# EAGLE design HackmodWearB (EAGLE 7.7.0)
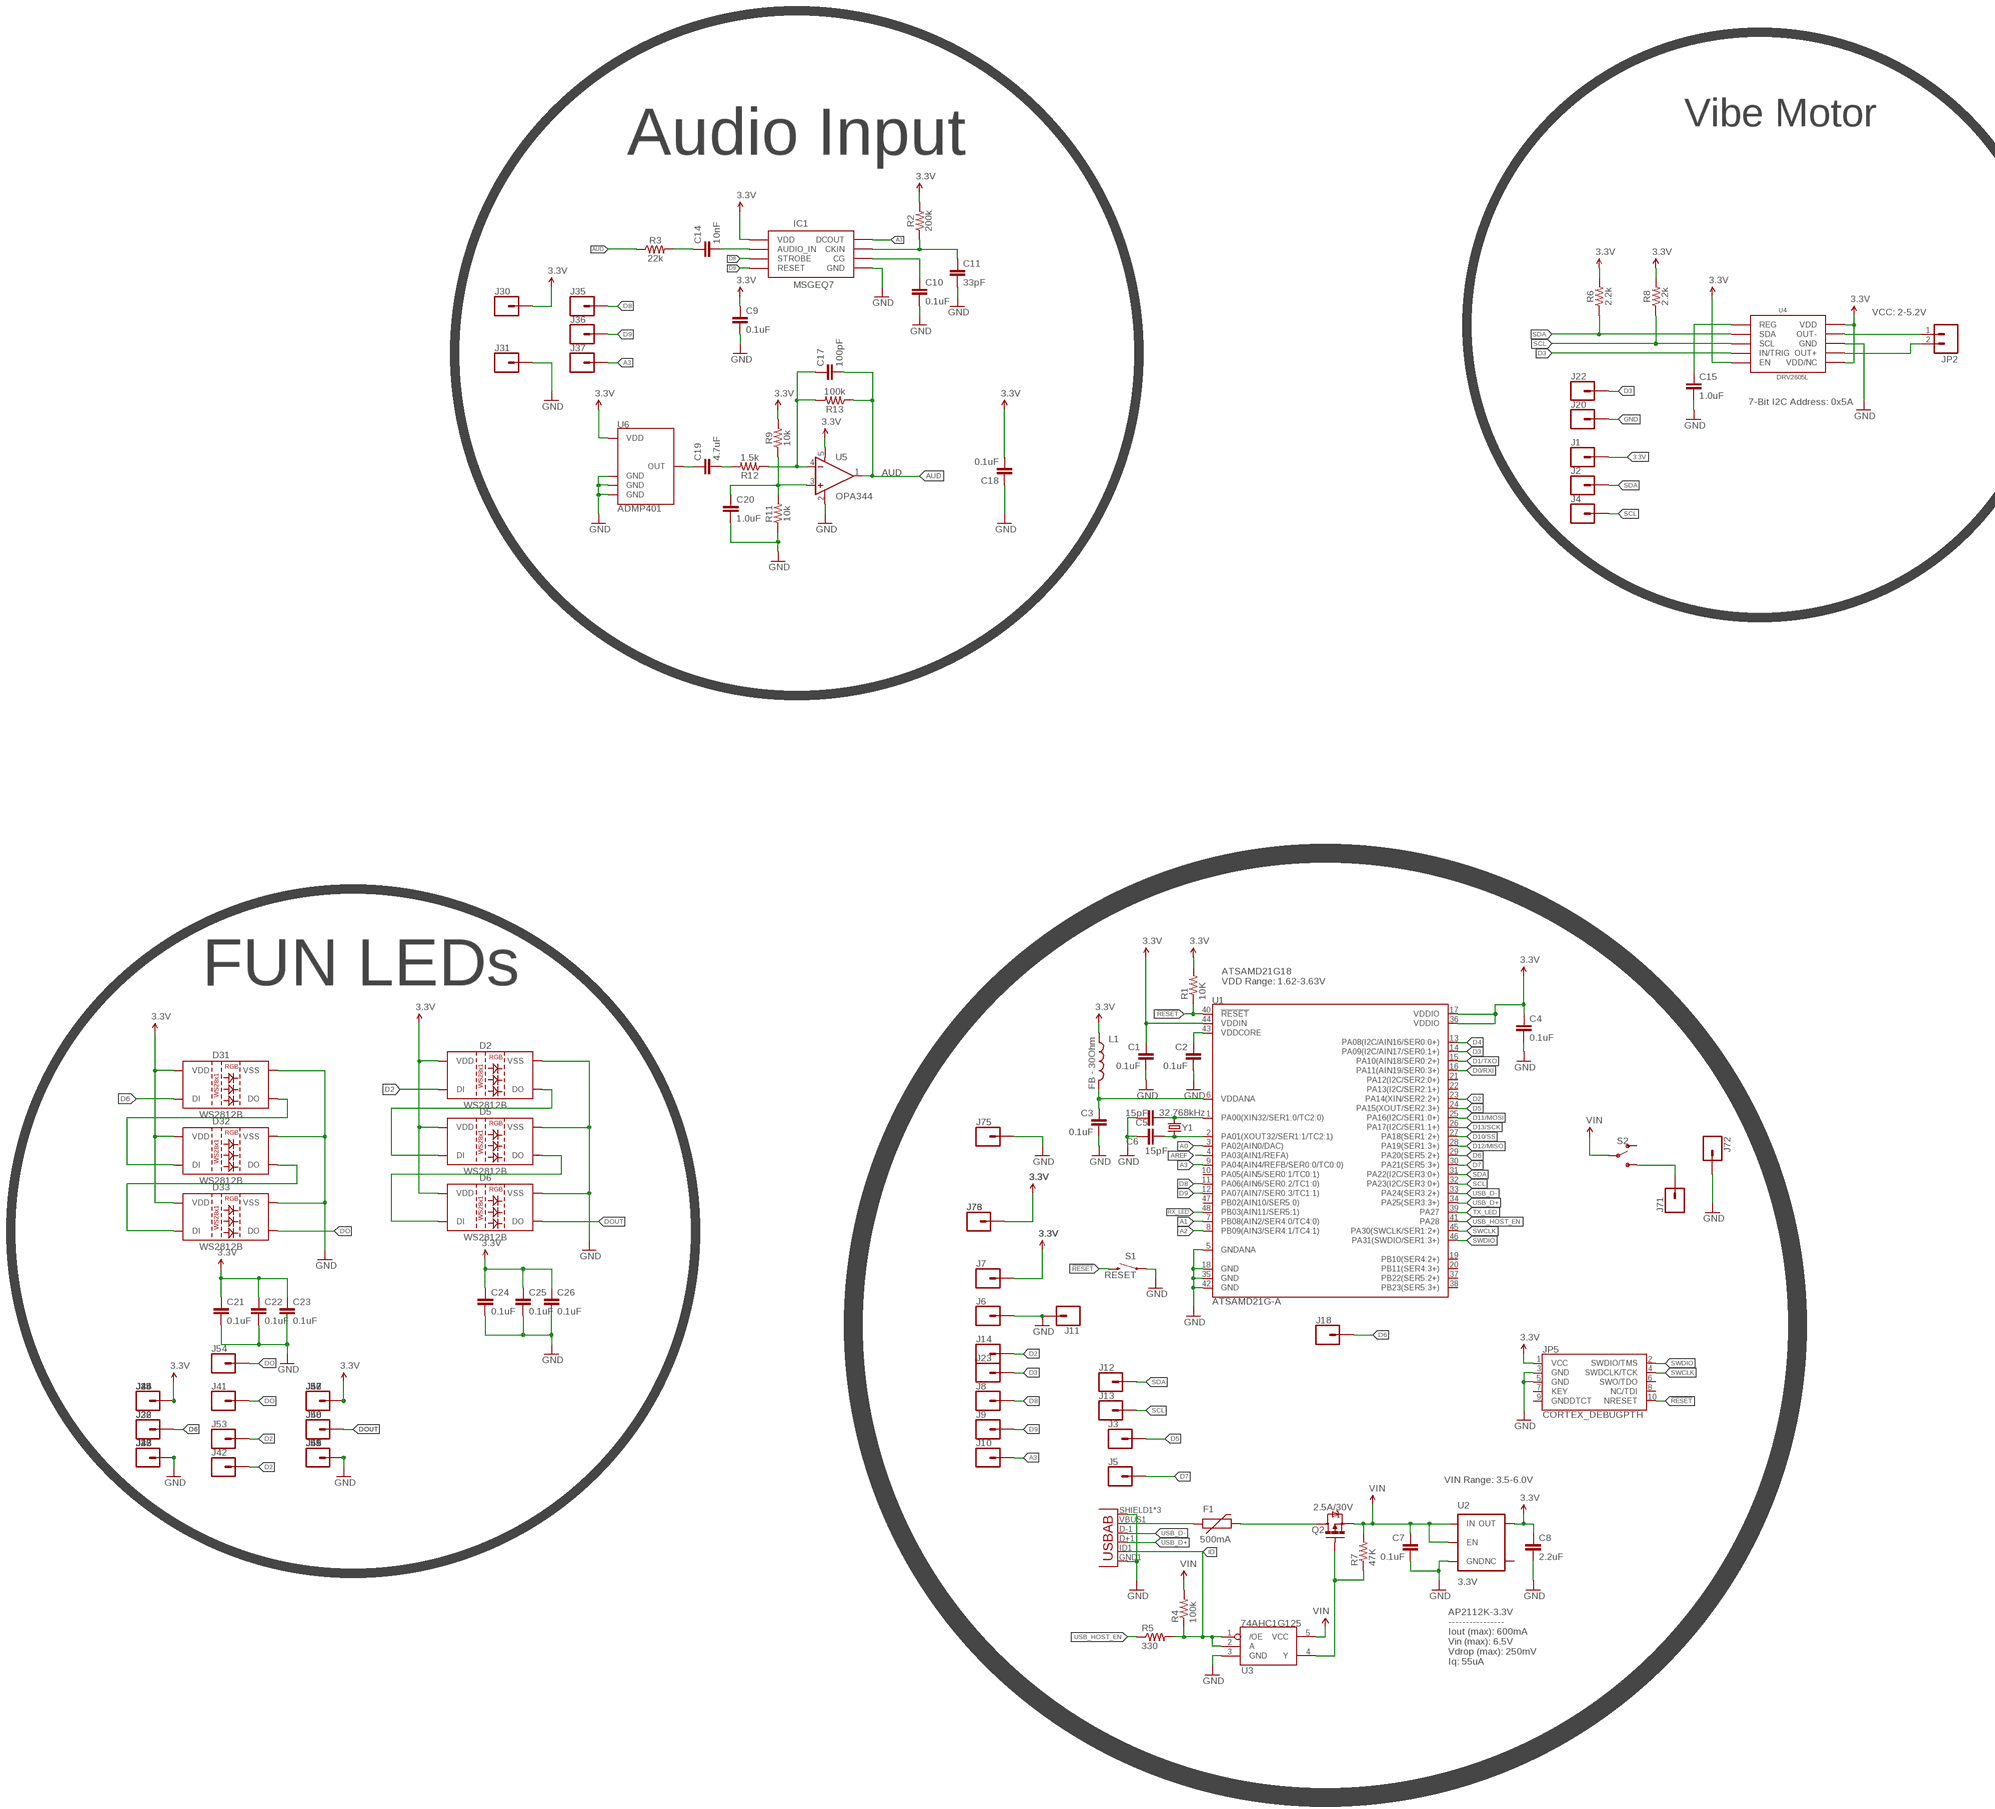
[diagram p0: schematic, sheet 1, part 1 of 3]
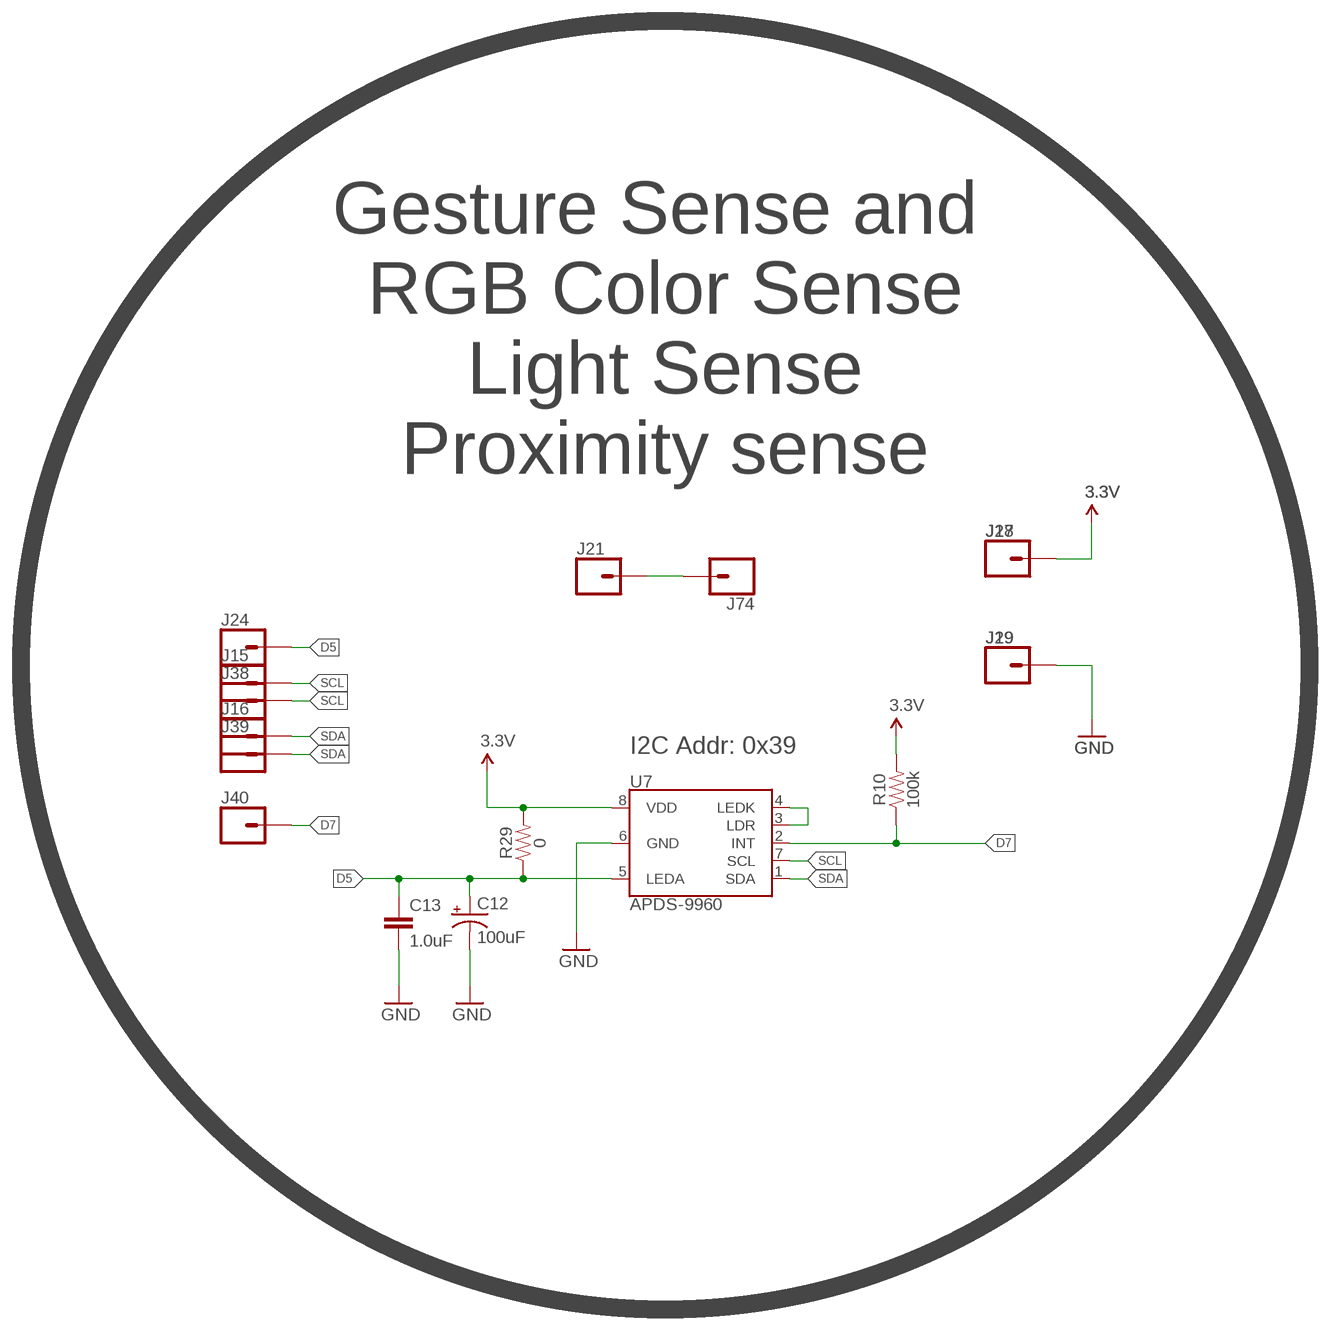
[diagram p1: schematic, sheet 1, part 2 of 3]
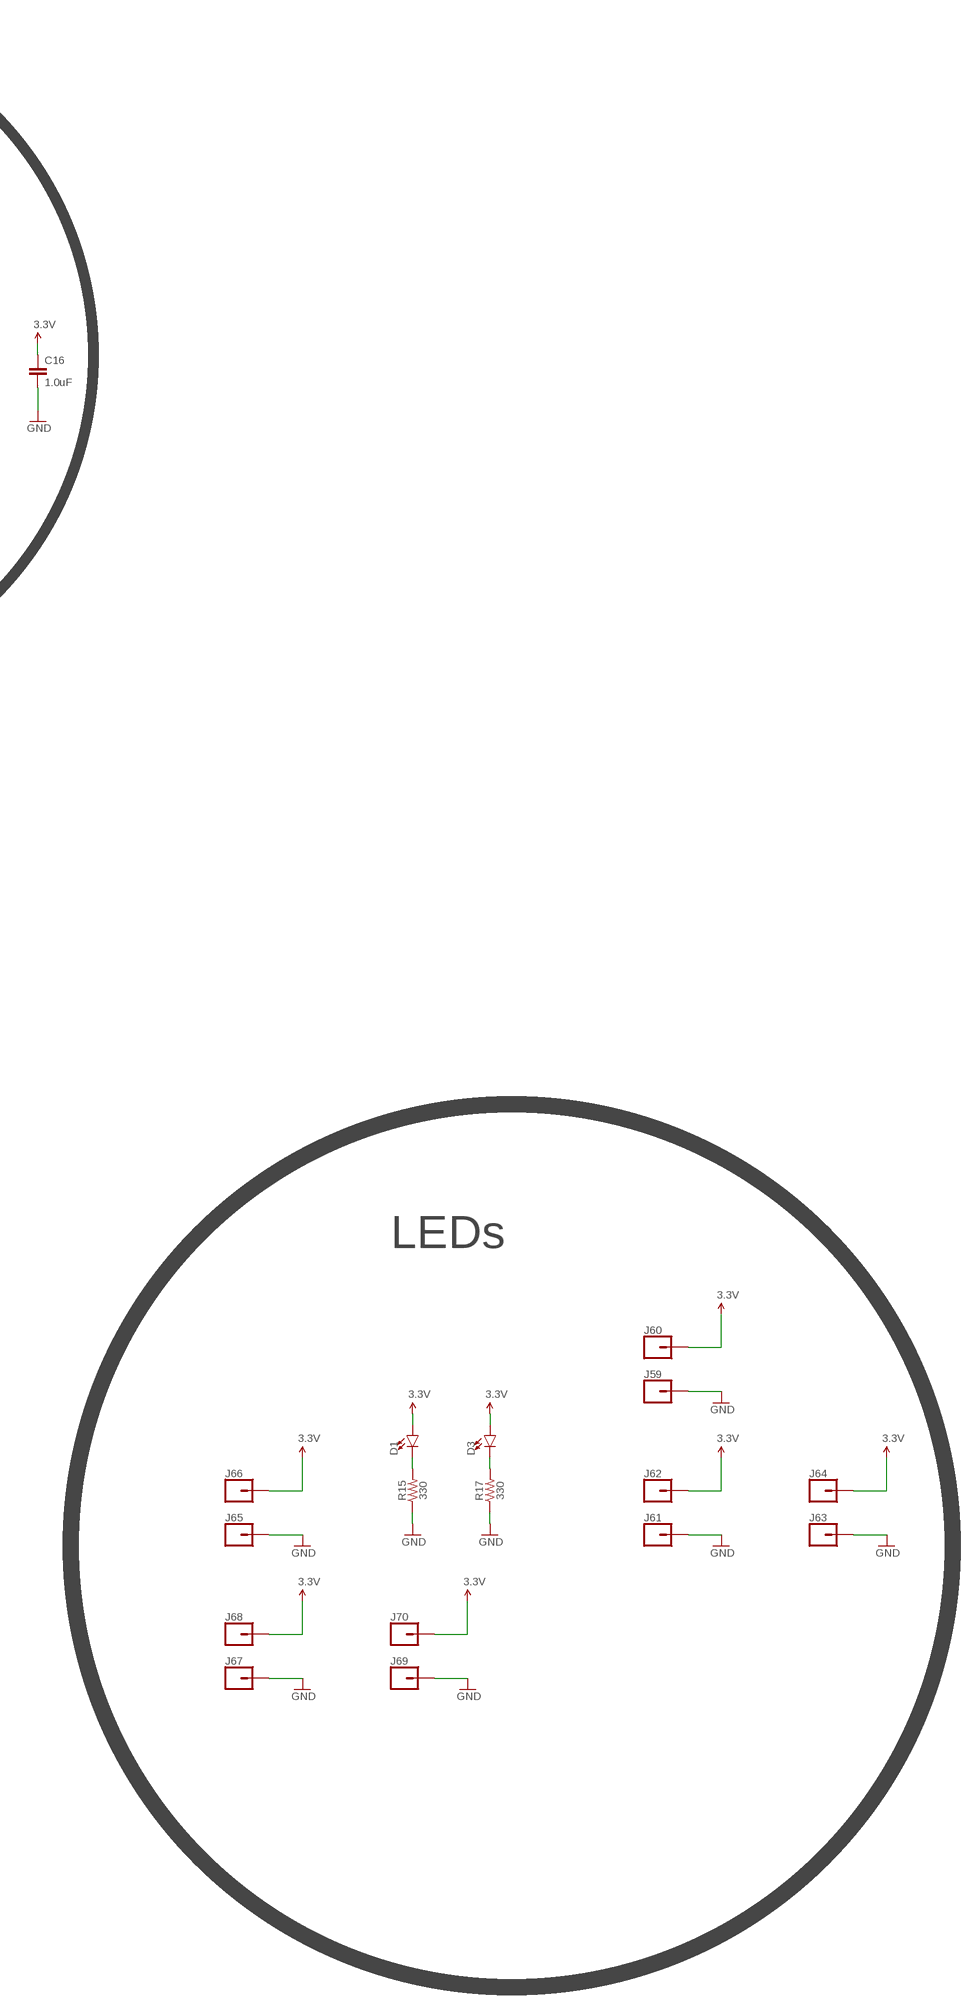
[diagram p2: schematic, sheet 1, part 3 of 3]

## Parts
C1  0.1uF  0.1UF-0603-25V-(+80/-20%)  [0603]
C2  0.1uF  0.1UF-0603-25V-(+80/-20%)  [0603]
C3  0.1uF  0.1UF-0603-25V-(+80/-20%)  [0603]
C4  0.1uF  0.1UF-0603-25V-(+80/-20%)  [0603]
C5  15pF  15PF-0603-50V-5%  [0603]
C6  15pF  15PF-0603-50V-5%  [0603]
C7  0.1uF  0.1UF-0603-25V-(+80/-20%)  [0603]
C8  2.2uF  2.2UF-10V-20%(0603)  [0603-CAP]
C9  0.1uF  0.1UF-0603-25V-(+80/-20%)  [0603]
C10  0.1uF  0.1UF-0603-25V-(+80/-20%)  [0603]
C11  33pF  33PF-0603-50V-5%  [0603]
C12  100uF  100UF-POLAR-EIA7343-10V-10%(TANT)  [EIA7343]
C13  1.0uF  1.0UF-0603-16V-10%  [0603]
C14  10nF  10NF-0603-50V-10%  [0603]
C15  1.0uF  1.0UF-16V-10%(0402)  [0402-CAP]
C16  1.0uF  1.0UF-16V-10%(0402)  [0402-CAP]
C17  100pF  100PF-0603-50V-5%  [0603]
C18  0.1uF  0.1UF-0603-25V-(+80/-20%)  [0603]
C19  4.7uF  4.7UF0603  [0603]
C20  1.0uF  1.0UF-0603-16V-10%  [0603]
C21  0.1uF  0.1UF-0603-25V-(+80/-20%)  [0603]
C22  0.1uF  0.1UF-0603-25V-(+80/-20%)  [0603]
C23  0.1uF  0.1UF-0603-25V-(+80/-20%)  [0603]
C24  0.1uF  0.1UF-0603-25V-(+80/-20%)  [0603]
C25  0.1uF  0.1UF-0603-25V-(+80/-20%)  [0603]
C26  0.1uF  0.1UF-0603-25V-(+80/-20%)  [0603]
D1  LED1206  [LED-1206]
D2  WS2812B  [WS2812B]
D3  LED1206  [LED-1206]
D5  WS2812B  [WS2812B]
D6  WS2812B  [WS2812B]
D31  WS2812B  [WS2812B]
D32  WS2812B  [WS2812B]
D33  WS2812B  [WS2812B]
F1  500mA  PTCSMD  [PTC-1206]
IC1  MSGEQ7P  MSGEQ7DIL  [DIP08]
J1  CONN_01  [1X01]
J2  CONN_01  [1X01]
J3  CONN_01  [1X01]
J4  CONN_01  [1X01]
J5  CONN_01  [1X01]
J6  CONN_01  [1X01]
J7  CONN_01  [1X01]
J8  CONN_01  [1X01]
J9  CONN_01  [1X01]
J10  CONN_01  [1X01]
J11  CONN_01  [1X01]
J12  CONN_01  [1X01]
J13  CONN_01  [1X01]
J14  CONN_01  [1X01]
J15  CONN_01  [1X01]
J16  CONN_01  [1X01]
J17  CONN_01  [1X01]
J18  CONN_01  [1X01]
J19  CONN_01  [1X01]
J20  CONN_01  [1X01]
J21  CONN_01  [1X01]
J22  CONN_01  [1X01]
J23  CONN_01  [1X01]
J24  CONN_01  [1X01]
J25  CONN_01  [1X01]
J26  CONN_01  [1X01]
J27  CONN_01  [1X01]
J28  CONN_01  [1X01]
J29  CONN_01  [1X01]
J30  CONN_01  [1X01]
J31  CONN_01  [1X01]
J32  CONN_01  [1X01]
J33  CONN_01  [1X01]
J34  CONN_01  [1X01]
J35  CONN_01  [1X01]
J36  CONN_01  [1X01]
J37  CONN_01  [1X01]
J38  CONN_01  [1X01]
J39  CONN_01  [1X01]
J40  CONN_01  [1X01]
J41  CONN_01  [1X01]
J42  CONN_01  [1X01]
J43  CONN_01  [1X01]
J44  CONN_01  [1X01]
J45  CONN_01  [1X01]
J46  CONN_01  [1X01]
J47  CONN_01  [1X01]
J48  CONN_01  [1X01]
J49  CONN_01  [1X01]
J50  CONN_01  [1X01]
J51  CONN_01  [1X01]
J52  CONN_01  [1X01]
J53  CONN_01  [1X01]
J54  CONN_01  [1X01]
J55  CONN_01  [1X01]
J56  CONN_01  [1X01]
J57  CONN_01  [1X01]
J58  CONN_01  [1X01]
J59  CONN_01  [1X01]
J60  CONN_01  [1X01]
J61  CONN_01  [1X01]
J62  CONN_01  [1X01]
J63  CONN_01  [1X01]
J64  CONN_01  [1X01]
J65  CONN_01  [1X01]
J66  CONN_01  [1X01]
J67  CONN_01  [1X01]
J68  CONN_01  [1X01]
J69  CONN_01  [1X01]
J70  CONN_01  [1X01]
J71  CONN_01  [1X01]
J72  CONN_01  [1X01]
J73  CONN_01  [1X01]
J74  CONN_01  [1X01]
J75  CONN_01  [1X01]
J76  CONN_01  [1X01]
JP2  M02PTH  [1X02@1]
JP3  USB-ABCONN-11794  [USB-AB-MICRO-SMD_V03]
JP5  CORTEX_DEBUGPTH  [2X5-PTH-1.27MM]
L1  FB - 30Ohm  INDUCTOR0603  [0603]
Q2  2.5A/30V  MOSFET-PCHANNELDMG2307L  [SOT23-3]
R1  10K  10KOHM-1/10W-1%(0603)0603  [0603-RES@1]
R2  200k  200KOHM-0603-1/10W-1%  [0603]
R3  22k  22KOHM-0603-1/10W-1%  [0603]
R4  100k  100KOHM-1/10W-1%(0603)  [0603-RES@1]
R5  330  330OHM1/10W1%(0603)  [0603-RES@1]
R6  2.2k  2.2KOHM-0603-1/10W-1%  [0603]
R7  47K  47KOHM1/10W1%(0603)  [0603-RES@1]
R8  2.2k  2.2KOHM-0603-1/10W-1%  [0603]
R9  10k  10KOHM-0603-1/10W-1%  [0603]
R10  100k  100KOHM-0603-1/10W-1%  [0603]
R11  10k  10KOHM-0603-1/10W-1%  [0603]
R12  1.5k  1.5KOHM-0603-1/10W-1%  [0603]
R13  100k  100KOHM-0603-1/10W-1%  [0603]
R15  330  330OHM-0603-1/10W-1%  [0603]
R17  330  330OHM-0603-1/10W-1%  [0603]
R29  0  0OHM-0603-1/10W-5%  [0603]
S1  RESET  SWITCH-MOMENTARY-2SMD-4.6X2.8MM  [TACTILE_SWITCH_SMD_4.6X2.8MM]
S2  SWITCH-SPDT-SMD-RIGHT-ANGLE  [SWITCH_SPST_SMD_A]
U1  ATSAMD21G-A  [TQFP-48]
U2  3.3V  V_REG_AP2112K-3.3V  [SOT23-5]
U3  74AHC1G125  [SOT23-5]
U4  DRV2605L  [VSSOP-10]
U5  OPA344  [SOT23-5]
U6  ADMP401  [ADMP401]
U7  APDS-9960  [APDS-9960]
Y1  32.768kHz  CRYSTAL3.2X1.5MM  [CRYSTAL-SMD-3.2X1.5MM]

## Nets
3.3V: C1.1 C4.1 C8.1 C9.1 C16.1 C18.2 C21.1 C22.1 C23.1 C24.1 C25.1 C26.1 D1.A D2.1(VDD) D3.A D5.1(VDD) D6.1(VDD) D31.1(VDD) D32.1(VDD) D33.1(VDD) IC1.1(VDD) J1.P$1 J7.P$1 J17.P$1 J25.P$1 J28.P$1 J30.P$1 J34.P$1 J44.P$1 J45.P$1 J47.P$1 J52.P$1 J56.P$1 J57.P$1 J60.P$1 J62.P$1 J64.P$1 J66.P$1 J68.P$1 J70.P$1 J73.P$1 J76.P$1 JP5.1(VCC) L1.1 R1.2 R2.2 R6.2 R8.2 R9.2 R10.2 R29.2 U1.17(VDDIO) U1.36(VDDIO) U1.44(VDDIN) U2.5(OUT) U4.P$5(EN) U4.P$6(VDD/NC) U4.P$10(VDD) U5.5(V+) U6.5(VDD) U7.8(VDD)
!RESET: JP5.10(NRESET) R1.1 S1.3 S1.4 U1.40(!RESET!)
A0: U1.3(PA02(AIN0/DAC))
A1: U1.7(PB08(AIN2/SER4:0/TC4:0))
A2: U1.8(PB09(AIN3/SER4:1/TC4:1))
A3: IC1.3(DCOUT) J10.P$1 J37.P$1 U1.9(PA04(AIN4/REFB/SER0:0/TC0:0))
AREF: U1.4(PA03(AIN1/REFA))
AUD: C17.2 R3.1 R13.1 U5.1(OUT)
D0/RXI: U1.16(PA11(AIN19/SER0:3+))
D1/TXO: U1.15(PA10(AIN18/SER0:2+))
D2: D2.4(DI) J14.P$1 J42.P$1 J53.P$1 U1.23(PA14(XIN/SER2:2+))
D3: J22.P$1 J23.P$1 U1.14(PA09(I2C/AIN17/SER0:1+)) U4.P$4(IN/TRIG)
D4: U1.13(PA08(I2C/AIN16/SER0:0+))
D5: C12.A(+) C13.1 J3.P$1 J24.P$1 R29.1 U1.24(PA15(XOUT/SER2:3+)) U7.5(LEDA)
D6: D31.4(DI) J18.P$1 J26.P$1 J32.P$1 U1.29(PA20(SER5:2+))
D7: J5.P$1 J40.P$1 R10.1 U1.30(PA21(SER5:3+)) U7.2(INT)
D8: IC1.4(STROBE) J8.P$1 J35.P$1 U1.11(PA06(AIN6/SER0:2/TC1:0))
D9: IC1.7(RESET) J9.P$1 J36.P$1 U1.12(PA07(AIN7/SER0:3/TC1:1))
D10/SS: U1.27(PA18(SER1:2+))
D11/MOSI: U1.25(PA16(I2C/SER1:0+))
D12/MISO: U1.28(PA19(SER1:3+))
D13/SCK: U1.26(PA17(I2C/SER1:1+))
DO: D33.2(DO) J41.P$1 J54.P$1
DOUT: D6.2(DO) J48.P$1 J50.P$1
GND: C1.2 C2.2 C3.2 C4.2 C5.1 C6.2 C7.2 C8.2 C9.2 C10.2 C11.2 C12.C(-) C13.2 C15.2 C16.2 C18.1 C20.2 C21.2 C22.2 C23.2 C24.2 C25.2 C26.2 D2.3(VSS) D5.3(VSS) D6.3(VSS) D31.3(VSS) D32.3(VSS) D33.3(VSS) IC1.2(GND) J6.P$1 J11.P$1 J19.P$1 J20.P$1 J27.P$1 J29.P$1 J31.P$1 J33.P$1 J43.P$1 J46.P$1 J49.P$1 J51.P$1 J55.P$1 J58.P$1 J59.P$1 J61.P$1 J63.P$1 J65.P$1 J67.P$1 J69.P$1 J72.P$1 J75.P$1 JP3.GND1(GND) JP3.SHIELD1(SHIELD) JP3.SHIELD2(SHIELD) JP3.SHIELD3(SHIELD) JP5.3(GND) JP5.5(GND) R11.1 R15.1 R17.1 S1.1 S1.2 U1.5(GNDANA) U1.18(GND) U1.35(GND) U1.42(GND) U2.2(GND) U3.3(GND) U4.P$8(GND) U5.2(V-) U6.2(GND) U6.4(GND) U6.6(GND) U7.6(GND)
ID: JP3.ID1(USBID) R4.1 R5.2 U3.1(/OE) U3.2(A)
N$1: F1.1 JP3.VBUS1(VBUS)
N$2: C5.2 U1.1(PA00(XIN32/SER1:0/TC2:0)) Y1.P$2
N$3: C19.1 U6.1(OUT)
N$4: C6.1 U1.2(PA01(XOUT32/SER1:1/TC2:1)) Y1.P$1
N$5: U7.3(LDR) U7.4(LEDK)
N$6: C17.1 R12.1 R13.2 U5.4(-IN)
N$7: F1.2 Q2.3(D)
N$8: J21.P$1 J74.P$1
N$9: Q2.1(G) R7.1 U3.4(Y)
N$10: C19.2 R12.2
N$11: C20.1 R9.1 R11.2 U5.3(+IN)
N$12: D1.C R15.2
N$13: C15.1 U4.P$1(REG)
N$14: D31.2(DO) D32.4(DI)
N$15: D3.C R17.2
N$16: D32.2(DO) D33.4(DI)
N$17: C14.2 IC1.5(AUDIO_IN)
N$18: C14.1 R3.2
N$19: C10.1 IC1.6(CG)
N$20: C11.1 IC1.8(CKIN) R2.1
N$21: J71.P$1 S2.3(S)
N$22: D2.2(DO) D5.4(DI)
N$23: D5.2(DO) D6.4(DI)
N$24: JP2.1 U4.P$9(OUT-)
N$25: JP2.2 U4.P$7(OUT+)
RX_LED: U1.48(PB03(AIN11/SER5:1))
SCL: J4.P$1 J13.P$1 J15.P$1 J38.P$1 R8.1 U1.32(PA23(I2C/SER3:0+)) U4.P$2(SCL) U7.7(SCL)
SDA: J2.P$1 J12.P$1 J16.P$1 J39.P$1 R6.1 U1.31(PA22(I2C/SER3:0+)) U4.P$3(SDA) U7.1(SDA)
SWCLK: JP5.4(SWDCLK/TCK) U1.45(PA30(SWCLK/SER1:2+))
SWDIO: JP5.2(SWDIO/TMS) U1.46(PA31(SWDIO/SER1:3+))
TX_LED: U1.39(PA27)
USB_D+: JP3.D+1(D+) U1.34(PA25(SER3:3+))
USB_D-: JP3.D-1(D-) U1.33(PA24(SER3:2+))
USB_HOST_EN: R5.1 U1.41(PA28)
VDDANA: C3.1 L1.2 U1.6(VDDANA)
VDDCORE: C2.1 U1.43(VDDCORE)
VIN: C7.1 Q2.2(S) R4.2 R7.2 S2.2(P) U2.1(IN) U2.3(EN) U3.5(VCC)
Unconnected: JP5.6(SWO/TDO) JP5.7(KEY) JP5.8(NC/TDI) JP5.9(GNDDTCT) S2.1(O) U1.10(PA05(AIN5/SER0:1/TC0:1)) U1.19(PB10(SER4:2+)) U1.20(PB11(SER4:3+)) U1.21(PA12(I2C/SER2:0+)) U1.22(PA13(I2C/SER2:1+)) U1.37(PB22(SER5:2+)) U1.38(PB23(SER5:3+)) U1.47(PB02(AIN10/SER5:0)) U2.4(NC)

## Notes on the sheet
- Vibe Motor
- Audio Input
- VCC: 2-5.2V
- 7-Bit I2C Address: 0x5A
- ATSAMD21G18
  VDD Range: 1.62-3.63V
- FUN LEDs
- LEDs
- VIN Range: 3.5-6.0V
- AP2112K-3.3V
  ----------------
  Iout (max): 600mA 
  Vin (max): 6.5V
  Vdrop (max): 250mV
  Iq: 55uA
- Gesture Sense and 
  RGB Color Sense
  Light Sense
  Proximity sense
- I2C Addr: 0x39

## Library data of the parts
C1-C4 C7 C9 C10 C18 C21-C26 = SparkFun-Capacitors:0.1UF: 0.1µF ceramic capacitors; PROD_ID: CAP-00810
C5 C6 = SparkFun-Capacitors:15PF: 15pF ceramic capacitors; PROD_ID: CAP-07881
C8 = SparkFun-Capacitors:2.2UF-10V-20%(0603): CAP-07888; PROD_ID: CAP-07888
C11 = SparkFun-Capacitors:33PF: 33pF ceramic capacitors; PROD_ID: CAP-10142
C12 = SparkFun-Capacitors:100UF-POLAR: 100µF polarized capacitors; PROD_ID: CAP-07890
C13 C20 = SparkFun-Capacitors:1.0UF: 1µF ceramic capacitors; PROD_ID: CAP-00868
C14 = SparkFun-Capacitors:10NF: 0.01uF/10nF/10,000pF ceramic capacitors; PROD_ID: CAP-00867
C15 C16 = SparkFun-Capacitors:1.0UF-16V-10%(0402); PROD_ID: CAP-12417
C17 = SparkFun-Capacitors:100PF: 100pF/0.1nF ceramic capacitors; PROD_ID: CAP-07883
C19 = SparkFun-Capacitors:4.7UF: 4.7µF ceramic capacitors; PROD_ID: CAP-08280
D1 D3 = SparkFun-LED:LED: LED (Generic)
D2 D5 D6 D31-D33 = SparkFun-LED:WS2812B: WS2812B SMD addressable RGB LED 5x5mm SMD LED with built-in controller IC. Color: Red/Green/Blue mC Rating: RGB: 390, 660, 180 mcd Forward Voltage: RGB: 2.0, 3.0, 3.0 V Packages:WS2812B SparkFun Products: Blynk Board - ESP8266; PROD_ID: DIO-12503
F1 = SparkFun-PowerIC:PTC: Resettable Fuse PTC; PROD_ID: RES-11150
IC1 = SparkFun-IC-Special-Function:MSGEQ7: 7-band graphic equalizer This IC is for making a 7 band/channel audio spectrometer. There are two versions of this part. The DIP available on the storefront, and the SO used in product. Datasheet SparkFun Products Storefront component: Graphic Equalizer Display Filter - MSGEQ7 (COM-10468) SparkFun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; PROD_ID: IC-12196
J1-J76 = SparkFun-Connectors:CONN_01: Single connection point. Often used as Generic Header-pin footprint for 0.1 inch spaced/style header connections
JP2 = SparkFun-Connectors:M02: Standard 2-pin 0.1" header. Use with
JP3 = SparkFun-Connectors:USB-AB: This is a USB AB connector that is compatible with USB OTG. i.e. this connector can serve as a host or device; PROD_ID: CONN-11794
JP5 = samd21-temp:CORTEX_DEBUG: Cortex Debug Connector Datasheet
L1 = SparkFun-Passives:INDUCTOR: Inductors; PROD_ID: RES-07859
Q2 = SparkFun-DiscreteSemi:MOSFET-PCHANNEL: Generic PMOSFET IRLML2244 - TRANS-11153 (SOT-23 -20V -4.3A) (1.Gate 2.Source 3.Drain) FQP27P06 - COM-10349 (TO-220 -60V -27A) (1.Gate 2.Source 3.Drain); PROD_ID: TRANS-11308
R1 = SparkFun-Resistors:10KOHM-1/10W-1%(0603): RES-00824; PROD_ID: RES-00824
R2 = SparkFun-Resistors:200KOHM: 200kΩ resistor; PROD_ID: RES-09385
R3 = SparkFun-Resistors:22KOHM: 22kΩ resistor; PROD_ID: RES-07853
R4 = SparkFun-Resistors:100KOHM-1/10W-1%(0603): RES-07828; PROD_ID: RES-07828
R5 = SparkFun-Resistors:330OHM1/10W1%(0603): RES-00818; PROD_ID: RES-00818
R6 R8 = SparkFun-Resistors:2.2KOHM: 2.2kΩ resistor; PROD_ID: RES-08272
R7 = SparkFun-Resistors:47KOHM1/10W1%(0603): RES-07871; PROD_ID: RES-07871
R9 R11 = SparkFun-Resistors:10KOHM: 10kΩ resistor; PROD_ID: RES-00824
R10 R13 = SparkFun-Resistors:100KOHM: 100kΩ resistor; PROD_ID: RES-07828
R12 = SparkFun-Resistors:1.5KOHM: 1.5kΩ resistor; PROD_ID: RES-08306
R15 R17 = SparkFun-Resistors:330OHM: 330Ω resistor; PROD_ID: RES-00818
R29 = SparkFun-Resistors:0OHM: 0Ω resistor; PROD_ID: RES-08609
S1 = samd21-temp:SWITCH-MOMENTARY-2: Various NO switches- pushbuttons, reed, etc; PROD_ID: SWCH-13065
S2 = SparkFun-Switches:SWITCH-SPDT: Single Pole, Double Throw (SPDT) Switch Single-pole, double-throw (SPDT) switch. Variant Overview SMD-AYZ0202 Surface Mount DPDT Switch (COM-00597) Used on e.g. LilyPad Arduino USB - ATmega32U4 Board PTH-11.6X4.0MM SPDT Mini Power Switch (COM-00102) Used on e.g. SparkFun Simon Says - Through-Hole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; PROD_ID: SWCH-10651; SF_SKU: COM-10860
U1 = samd21-temp:ATSAMD21G: Atmel SAMD21G SMART ARM-Based Microcontroller The Atmel ® | SMART ™ SAM D21 is a series of low-power microcontrollers using the 32-bit ARM ® Cortex ® -M0+ processor, and ranging from 32- to 64-pins with up to 256KB Flash and 32KB of SRAM. The SAM D21 devices operate at a maximum frequency of 48MHz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; PROD_ID: IC-13064
U2 = SparkFun-PowerIC:V_REG_AP2112: AP2112 - 600mA CMOS LDO Regulator w/ Enable The AP2112 is CMOS process low dropout linear regulator with enable function, the regulator delivers a guaranteed 600mA (min.) continuous load current. Features Output Voltage Accuracy: ±1.5% Output Current: 600mA (Min.) Foldback Short Current Protection: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; PROD_ID: VREG-12457
U3 = SparkFun-DigitalIC:74AHC1G125: Single bus buffer gate with 3-state output; PROD_ID: IC-11920
U4 = SparkFun-PowerIC:DRV2605L; PROD_ID: IC-13504
U5 = SparkFun:OPA344
U6 = SparkFun-Sensors:ADMP401: ADMP401 - Omnidirection Bottom-Port MEMS Microphone The ADMP401 is a high quality, low cost, low power analog output bottom-ported omnidirectional MEMS microphone. The ADMP401 consists of a MEMS microphone element, an impedance converter, and an output amplifier. The ADMP401 sensitivity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; PROD_ID: IC-09773
U7 = SparkFun-Sensors:APDS-9960: Avago APDS-9960 Digital Proximity, Ambient Light, RGB, and Gesture Sensor. The APDS-9960 offers ambient light and color measuring, proximity detection, and touchless gesture sensing. It features UV and IR blocking filters, four separate diodes sensitive to different directions, and an I2C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; PROD_ID: SEN-12005
Y1 = samd21-temp:CRYSTAL: Various standard crystals. Proven footprints.; PROD_ID: XTAL-13062

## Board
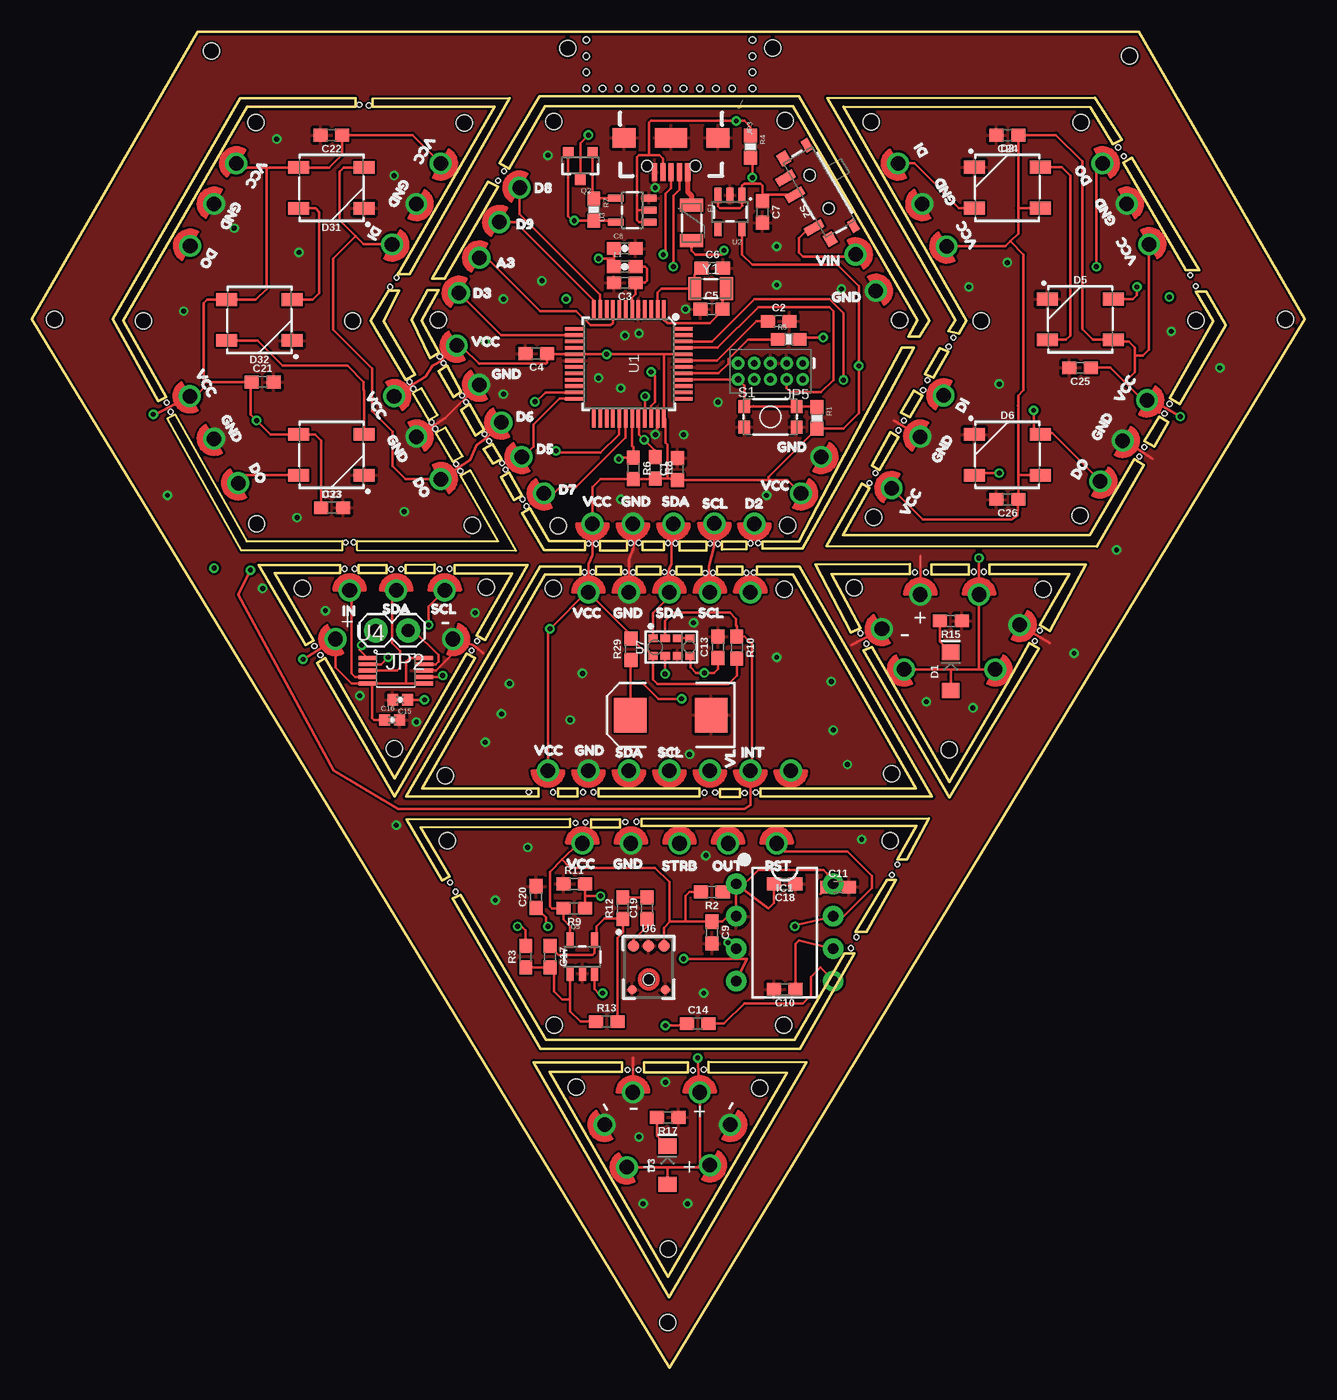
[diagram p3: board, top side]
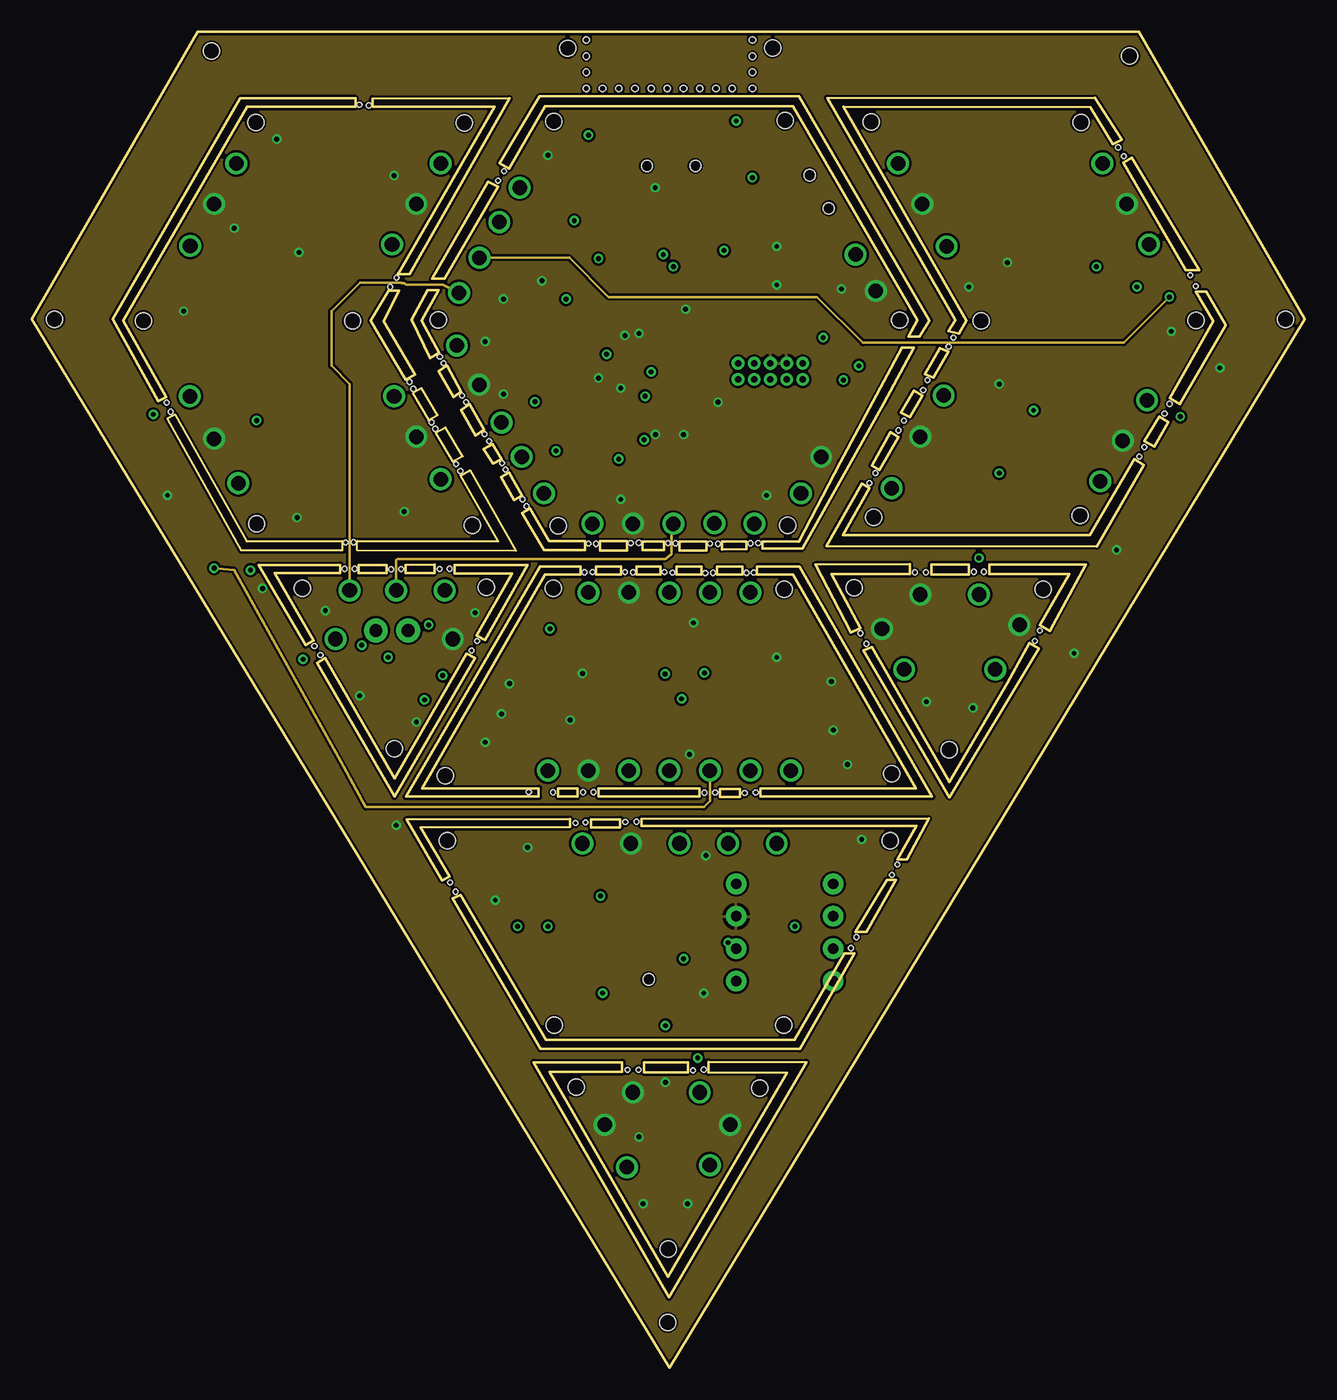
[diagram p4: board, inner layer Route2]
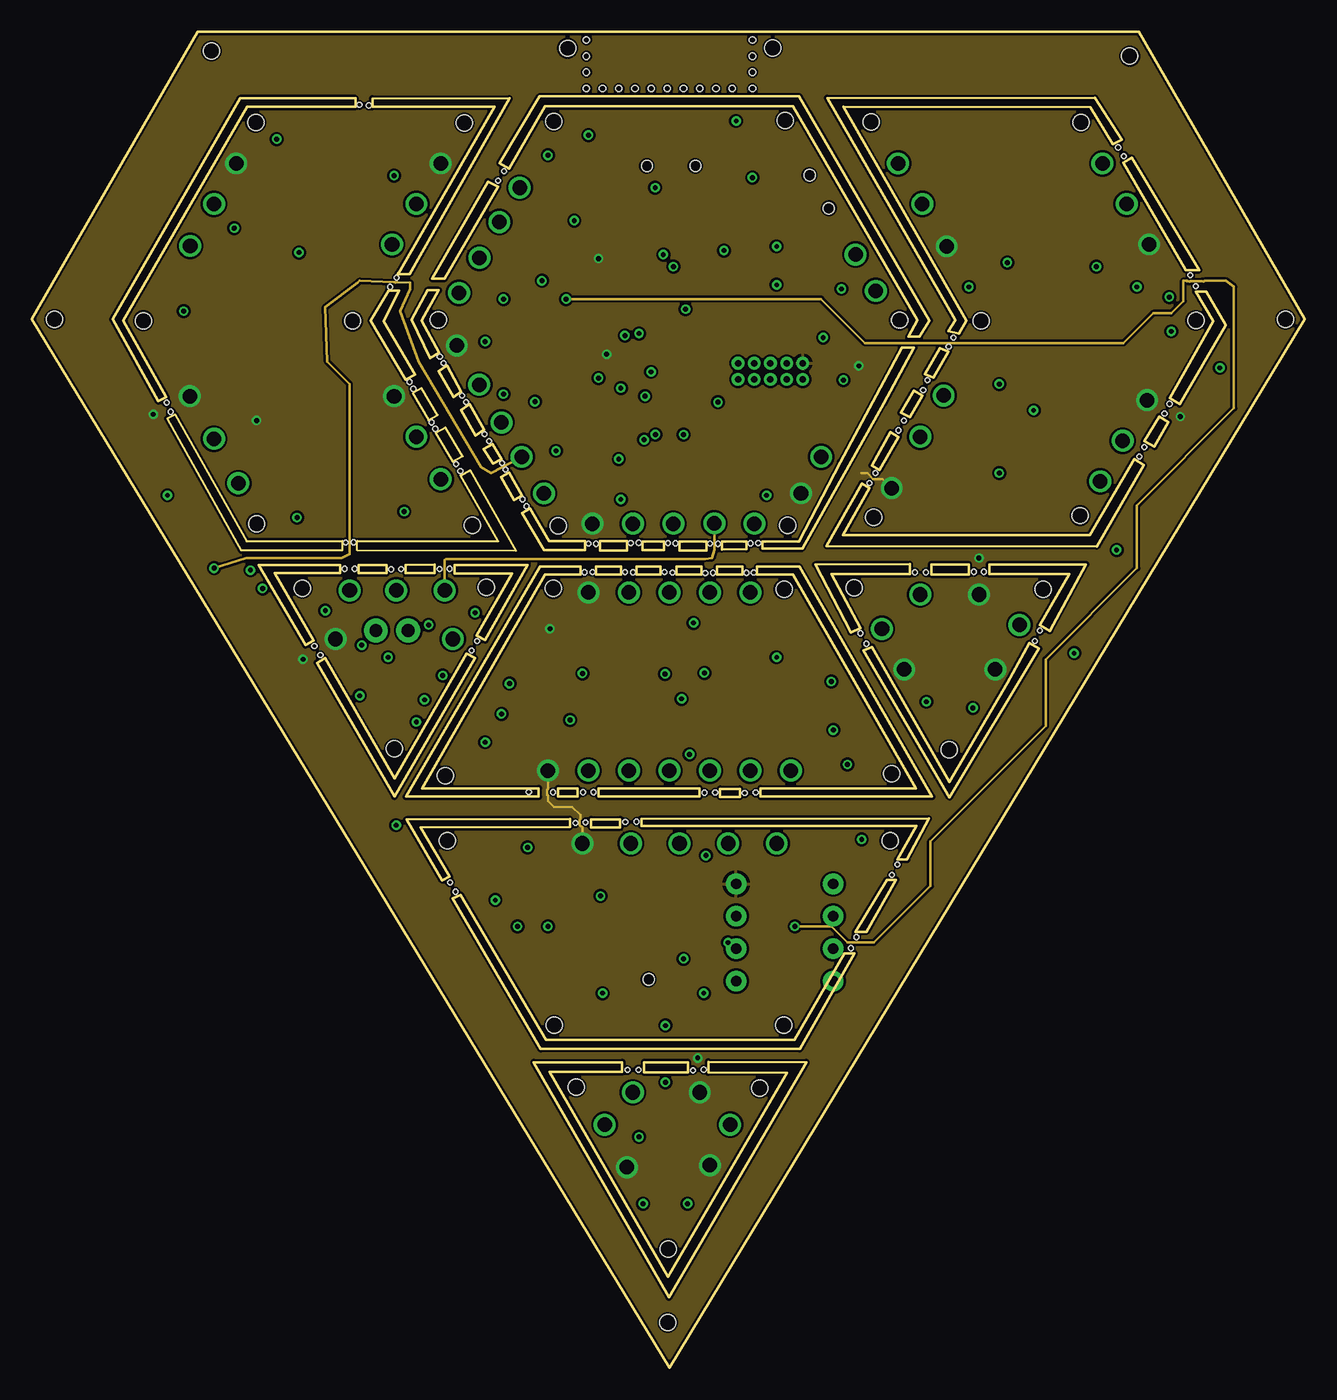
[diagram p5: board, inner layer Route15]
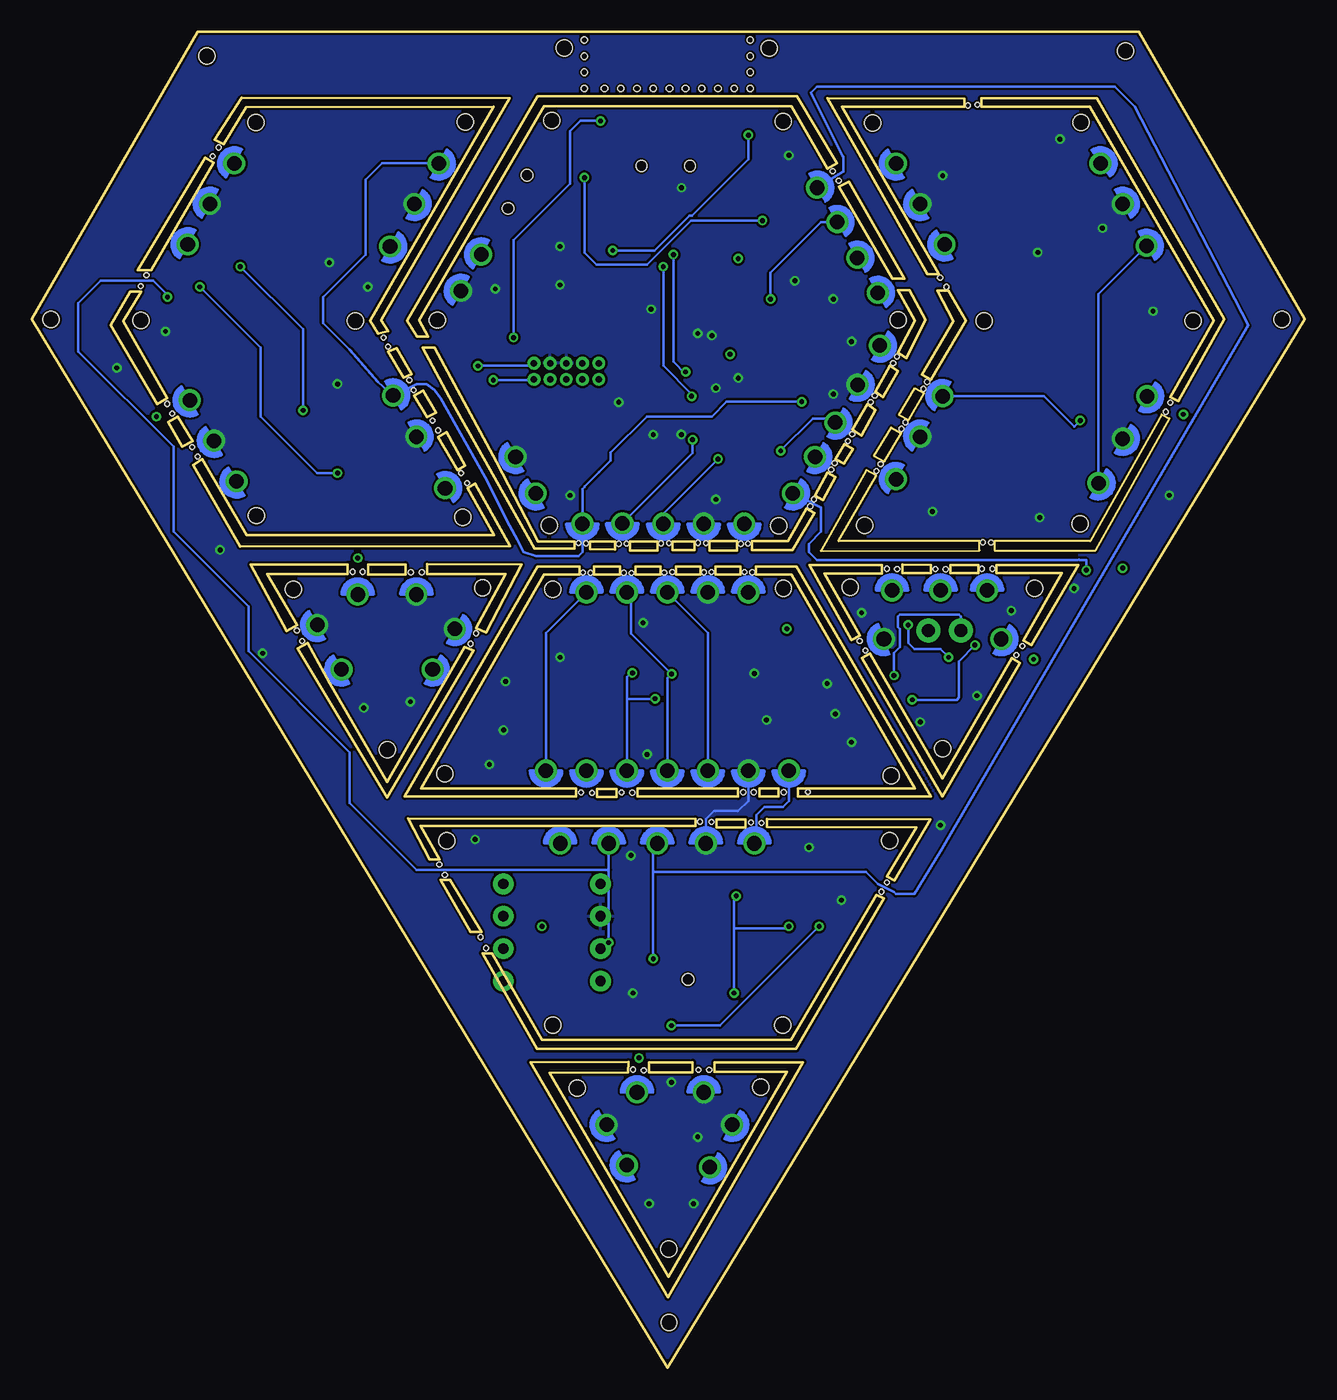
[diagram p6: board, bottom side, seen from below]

Size 99.85 x 104.77 mm. Coordinates in mm from the lower left corner, seen from the top.
Outline: 292 segments
Copper layers (1*2*15*16): Top 0.035559375mm / dielectric 0.47751875mm / Route2 0.035559375mm / dielectric 0.47751875mm / Route15 0.035559375mm / dielectric 0.47751875mm / Bottom 0.035559375mm
Design rules "SparkFun-4-layer-TIGHT": minimum track width 7mil, minimum drill 15mil, track to track 7mil, track to pad 7mil, pad to pad 7mil, via to via 7mil, smd to smd 7mil, copper to edge 7mil, drill to drill 7mil, minimum pad ring 7mil, minimum via ring 7mil, stop-mask expansion 4mil, vias tented up to drill 25mil, thermal gap 10mil
Holes 1.27 mm at 32.43,46.41 34.54,66.06 79.33,61.05 33.91,97.63 40.97,26.87 67.31,41.33 59.28,66.06 21.21,61.14 28.42,48.54 42.03,103.49 58.99,26.86 35.66,61.21 86.12,102.87 65.84,97.69 66.04,66.69 82.28,97.69 40.9,61.12 59,61.05 41.28,66.02 31.89,82.19 40.93,97.76 49.88,3.54 8.76,82.12 17.56,97.66 17.63,66.2 71.96,48.48 74.47,82.11 64.5,61.18 67.45,46.58 82.23,66.83 58.1,103.5 25.16,82.09 14.08,103.27 42.7,22 57.08,21.94 32.58,41.34 59.09,97.83 68.05,82.16 91.3,82.14 49.91,9.32 1.79,82.22 98.34,82.23
Holes 0.51 mm at 43.5,100.33 43.5,101.6 43.5,102.87 43.5,104.14 56.52,100.33 56.52,101.6 56.52,102.87 56.52,104.14 48.58,100.33 47.31,100.33 46.04,100.33 44.77,100.33 53.66,100.33 52.39,100.33 51.12,100.33 49.85,100.33 54.93,100.33
Holes 0.38 mm at 25.69,99.05 26.43,99 28.61,85.49 28.11,84.77 29.63,77.32 29.92,76.78 31.34,74.15 31.65,73.64 33.27,70.89 33.6,70.33 32,79.29 32.3,78.78 33.74,76.23 34.06,75.72 35.51,73.23 35.85,72.66 36.88,70.96 37.16,70.43 38.49,68.1 38.8,67.56 43.68,64.65 44.25,64.62 46.98,64.67 47.6,64.7 49.89,64.69 50.5,64.66 53.2,64.64 53.82,64.62 56.38,64.66 56.97,64.67 56.05,62.35 56.62,62.38 53.43,62.35 52.82,62.34 50.25,62.36 49.62,62.4 47.14,62.39 46.53,62.41 43.97,62.4 43.35,62.39 24.61,64.73 25.25,64.74 24.52,62.66 25.32,62.66 28.18,62.62 28.97,62.64 31.98,62.64 32.78,62.66 34.93,56.99 34.48,56.25 22.16,56.6 22.63,55.89 38.98,45.15 40.88,45.13 43.23,45.13 44.06,45.13 52.76,45.09 53.61,45.1 55.92,45.07 56.78,45.1 42.63,42.72 43.43,42.77 46.55,42.79 47.43,42.82 32.79,38.07 33.22,37.33 67.46,38.64 67.89,39.47 64.67,33.76 64.24,32.9 51.85,23.32 52.71,23.37 46.72,23.35 47.57,23.36 65,57.6 65.46,56.78 79.07,57.8 78.66,57 74.69,62.43 73.9,62.43 70.13,62.39 69.27,62.39 87.27,72.21 86.86,71.47 89.24,75.6 88.85,74.83 91.31,84.82 90.87,85.68 85.66,95.03 85.2,95.71 72.28,80.8 71.91,80.08 70.24,77.45 69.91,76.69 68.41,74.29 67.98,73.51 66.18,70.17 65.71,69.37 36.56,93.1 37.03,93.83 10.57,75.7 10.9,74.97

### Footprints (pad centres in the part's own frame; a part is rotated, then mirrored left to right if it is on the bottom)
0603 = smd 1.1 x 1: 1 -0.85,0; 2 0.85,0
0603-CAP = smd 1.1 x 1: 1 -0.85,0; 2 0.85,0
EIA7343 = smd 2.55 x 2.7: A 3.17,0; C -3.17,0
0402-CAP = smd 0.85 x 0.9: 1 -0.58,0; 2 0.58,0
LED-1206 = smd 1.2 x 1.4: A -1.5,0; C 1.5,0
WS2812B = smd 1.651 x 1: 1 2.577,-1.6; 2 2.577,1.6; 3 -2.577,1.6; 4 -2.577,-1.6
PTC-1206 = smd 1 x 1.8: 1 -1.4,0; 2 1.4,0
DIP08 = drill 0.813 pad 1.626: 1 -3.81,-3.81; 2 -1.27,-3.81; 3 1.27,-3.81; 4 3.81,-3.81; 5 3.81,3.81; 6 1.27,3.81; 7 -1.27,3.81; 8 -3.81,3.81
1X01 = drill 1.143: P$1 0,0
1X02@1 = drill 1.016 pad 1.88: 1 0,0; 2 2.54,0
USB-AB-MICRO-SMD_V03 = smd 1.4 x 0.4: D+1 2.7,0; D-1 2.7,0.65; GND1 2.7,-1.3; ID1 2.7,-0.65; VBUS1 2.7,1.3 | smd 1.5 x 1.8: SHIELD1 0,3.68; SHIELD3 0,-3.68 | smd 1.5 x 2.5: SHIELD2 0,0 | hole 0.85: 2.2,1.9; 2.2,-1.9
2X5-PTH-1.27MM = drill 0.508 pad 1: 1 -2.54,-0.635; 2 -2.54,0.635; 3 -1.27,-0.635; 4 -1.27,0.635; 5 0,-0.635; 6 0,0.635; 7 1.27,-0.635; 8 1.27,0.635; 9 2.54,-0.635; 10 2.54,0.635
SOT23-3 = smd 0.8 x 0.9: 1 -0.95,-1; 2 0.95,-1; 3 0,1.1
0603-RES@1 = smd 1.1 x 1: 1 -0.85,0; 2 0.85,0
TACTILE_SWITCH_SMD_4.6X2.8MM = smd 0.9 x 1: 1 -2.05,-0.8; 2 2.05,-0.8; 3 2.05,0.8; 4 -2.05,0.8
SWITCH_SPST_SMD_A = smd 0.7 x 1.5: 1 -2.25,-1.75; 2 -0.75,-1.75; 3 2.25,-1.75 | smd 1 x 0.6: GND1 -3.65,1; GND3 3.65,1 | smd 1 x 0.8: GND2 -3.65,-1.1; GND4 3.65,-1.1 | hole 0.9: -1.5,0; 1.5,0
TQFP-48 = smd 1.5 x 0.28: 1 -4.25,2.75; 2 -4.25,2.25; 3 -4.25,1.75; 4 -4.25,1.25; 5 -4.25,0.75; 6 -4.25,0.25; 7 -4.25,-0.25; 8 -4.25,-0.75; 9 -4.25,-1.25; 10 -4.25,-1.75; 11 -4.25,-2.25; 12 -4.25,-2.75; 25 4.25,-2.75; 26 4.25,-2.25; 27 4.25,-1.75; 28 4.25,-1.25; 29 4.25,-0.75; 30 4.25,-0.25; 31 4.25,0.25; 32 4.25,0.75; 33 4.25,1.25; 34 4.25,1.75; 35 4.25,2.25; 36 4.25,2.75 | smd 0.28 x 1.5: 13 -2.75,-4.25; 14 -2.25,-4.25; 15 -1.75,-4.25; 16 -1.25,-4.25; 17 -0.75,-4.25; 18 -0.25,-4.25; 19 0.25,-4.25; 20 0.75,-4.25; 21 1.25,-4.25; 22 1.75,-4.25; 23 2.25,-4.25; 24 2.75,-4.25; 37 2.75,4.25; 38 2.25,4.25; 39 1.75,4.25; 40 1.25,4.25; 41 0.75,4.25; 42 0.25,4.25; 43 -0.25,4.25; 44 -0.75,4.25; 45 -1.25,4.25; 46 -1.75,4.25; 47 -2.25,4.25; 48 -2.75,4.25
SOT23-5 = smd 0.55 x 1.2: 1 -0.95,-1.3; 2 0,-1.3; 3 0.95,-1.3; 4 0.95,1.3; 5 -0.95,1.3
VSSOP-10 = smd 1.45 x 0.3: P$1 -1.905,1.06; P$2 -1.905,0.56; P$3 -1.905,0.06; P$4 -1.905,-0.44; P$5 -1.905,-0.94; P$6 2.495,-0.94; P$7 2.495,-0.44; P$8 2.495,0.06; P$9 2.495,0.56; P$10 2.495,1.06
ADMP401 = smd 0.9 x 0.9: 1 -1.2,2.62; 5 1.2,2.62; 6 0,2.62 | smd 0.7 x 0.7: 2 1.3,-0.8; 4 -1.3,-0.8 | hole 0.9: 0,0
APDS-9960 = smd 0.6 x 0.72: 1 0.7,1.455; 2 0.7,0.485; 3 0.7,-0.485; 4 0.7,-1.455; 5 -0.7,-1.455; 6 -0.7,-0.485; 7 -0.7,0.485; 8 -0.7,1.455
CRYSTAL-SMD-3.2X1.5MM = smd 1 x 1.8: P$1 -1.25,0; P$2 1.25,0

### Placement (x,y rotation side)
C1  50.64,70.48 90 top
C2  58.58,82.07 0 top
C3  46.51,85.09 180 top
C4  39.56,79.53 180 top
C5  53.31,83.02 0 top
C6  53.37,86.24 0 top
C7  57.31,90.65 270 top
C8  46.51,87.79 0 top
C9  53.34,34.13 270 top
C10  59.05,29.69 180 top
C11  63.25,37.69 0 top
C12  50.11,51.19 180 top
C13  53.82,56.52 90 top
C14  52.23,26.99 0 top
C15  28.89,52.39 180 top
C16  28.26,50.8 0 top
C17  40.64,32.23 270 top
C18  59.05,37.94 180 top
C19  48.26,36.04 90 top
C20  39.55,36.91 90 top
C21  18.1,77.31 0 top
C22  23.49,96.68 180 top
C23  23.55,67.45 0 top
C24  76.52,96.68 180 top
C25  82.23,78.42 180 top
C26  76.52,68.1 180 top
D1  72.07,54.61 90 top
D2  76.52,92.55 0 top
D3  49.85,15.88 90 top
D5  82.24,82.22 0 top
D6  76.52,71.6 0 top
D31  23.5,92.53 180 top
D32  17.85,82.17 180 top
D33  23.49,71.6 180 top
F1  51.75,89.79 270 top
IC1  59.05,34.13 270 top
J1  23.81,57.15 120 top
J2  28.57,60.96 0 top
J3  38.42,71.44 120 top
J4  32.39,60.96 0 top
J5  40.16,68.58 120 top
J6  35.08,77.1 120 top
J7  67.44,68.98 60 top
J8  38.26,92.55 60 top
J9  36.67,89.85 60 top
J10  35.11,87.05 60 top
J11  47.15,66.2 180 top
J12  50.32,66.2 180 top
J13  50.01,46.83 180 top
J14  56.67,66.2 180 top
J15  53.18,60.8 0 top
J16  50.01,60.8 0 top
J17  43.66,60.8 0 top
J18  36.83,74.14 120 top
J19  46.83,60.8 0 top
J20  33.02,57.15 250 top
J21  59.53,46.83 180 top
J22  24.92,60.96 0 top
J23  33.5,84.3 60 top
J24  53.18,46.83 180 top
J25  32.07,94.46 240 top
J26  32.07,69.69 300 top
J27  14.29,91.28 60 top
J28  40.48,46.83 180 top
J29  43.66,46.83 180 top
J30  43.18,41.12 0 top
J31  46.99,41.12 0 top
J32  28.26,88.11 240 top
J33  30.16,73.02 300 top
J34  28.42,76.2 300 top
J35  50.8,41.12 0 top
J36  58.42,41.12 0 top
J37  54.61,41.12 0 top
J38  53.54,66.23 180 top
J39  46.83,46.83 180 top
J40  56.36,46.83 180 top
J41  16.19,69.37 120 top
J42  71.52,76.25 60 top
J43  30.16,91.28 240 top
J44  16.03,94.46 55 top
J45  12.38,76.2 120 top
J46  14.29,72.87 120 top
J47  71.75,87.95 120 top
J48  83.98,94.46 300 top
J49  85.88,91.28 300 top
J50  83.8,69.52 240 top
J51  69.85,91.28 120 top
J52  87.63,88.11 300 top
J53  67.94,94.46 120 top
J54  12.42,87.99 60 top
J55  69.69,73.02 60 top
J56  33.34,80.17 120 top
J57  87.47,75.88 240 top
J58  85.57,72.71 240 top
J59  77.47,58.26 240 top
J60  75.56,54.77 240 top
J61  66.67,57.94 120 top
J62  68.42,54.77 120 top
J63  69.69,60.64 0 top
J64  74.3,60.64 0 top
J65  47.15,21.59 0 top
J66  53.18,15.88 240 top
J67  44.93,19.05 120 top
J68  46.67,15.72 120 top
J69  54.77,19.05 240 top
J70  52.39,21.59 0 top
J71  64.61,87.31 300 top
J72  66.2,84.45 300 top
J73  43.97,66.2 180 top
J74  56.36,60.8 0 top
J75  61.91,71.44 240 top
J76  60.33,68.58 240 top
JP2  29.52,57.83 180 top
JP3  50.15,96.46 270 top
JP5  57.93,78.15 180 top
L1  46.51,86.36 0 top
Q2  43.02,94.3 180 top
R1  61.58,74.49 270 top
R2  53.34,37.31 180 top
R3  38.73,32.23 90 top
R4  56.36,95.77 270 top
R5  59.37,80.64 0 top
R6  47.18,70.54 270 top
R7  44.09,90.83 270 top
R8  48.9,70.58 270 top
R9  42.55,36.04 180 top
R10  55.29,56.48 270 top
R11  42.55,37.94 0 top
R12  46.36,36.04 90 top
R13  45.09,27.15 0 top
R15  72.09,58.58 180 top
R17  49.89,19.63 180 top
R29  46.99,56.36 90 top
S1  57.93,74.57 0 top
S2  61.75,92.23 300 top
U1  46.83,78.74 270 top
U2  54.77,90.65 180 top
U3  47.1,90.79 90 top
U4  28.26,54.61 0 top
U5  43.18,32.23 0 top
U6  48.39,30.45 0 top
U7  50.16,56.52 90 top
U$1  [GND2]  45.56,67.94 0 top
U$2  [A313]  35.72,86.68 0 top
U$3  [D517]  38.89,72.07 0 top
U$4  [D314]  33.81,84.3 0 top
U$5  [DO7]  16.99,71.44 300 top
U$6  [D616]  37.31,74.61 0 top
U$7  [D718]  40.64,68.9 0 top
U$8  [D811]  38.73,92.55 0 top
U$9  [D912]  37.31,89.69 0 top
U$10  [GND2]  14.76,75.25 300 top
U$11  [DI6]  27.46,90.01 240 top
U$12  [GND2]  35.4,77.95 0 top
U$13  [SCL5]  51.91,67.79 0 top
U$14  [SDA4]  48.74,67.94 0 top
U$15  [STRB8]  48.74,39.37 0 top
U$16  [VCC1]  41.12,39.53 0 top
U$17  [RST9]  56.83,39.37 0 top
U$18  [OUT10]  52.71,39.37 0 top
U$19  [GND2]  44.93,39.53 0 top
U$20  [VCC1]  41.59,59.21 0 top
U$21  [GND2]  44.93,59.21 0 top
U$22  [SDA4]  48.26,59.21 0 top
U$23  [SCL5]  51.59,59.21 0 top
U$24  [SCL5]  48.42,48.26 0 top
U$25  [SDA4]  45.09,48.26 0 top
U$26  [GND2]  57.79,72.23 0 top
U$27  [INT23]  54.93,48.26 0 top
U$28  [VL22]  54.77,46.35 90 top
U$29  [GND2]  41.91,48.42 0 top
U$30  [VCC21]  38.58,48.42 0 top
U$31  [VCC1]  56.36,69.22 0 top
U$32  [VCC1]  42.39,67.94 0 top
U$33  [VCC1]  33.66,80.49 0 top
U$34  [D219]  55.25,67.79 0 top
U$35  [VCC1]  12.7,78.9 300 top
U$36  [VIN20]  60.8,86.84 0 top
U$37  [GND2]  62.07,83.98 0 top
U$38  [GND2]  62.07,83.98 0 top
U$39  [VCC1]  18.57,95.25 240 top
U$40  [GND2]  29.69,93.66 240 top
U$41  [VCC1]  31.75,97.16 240 top
U$42  [GND2]  16.51,91.92 240 top
U$43  [DO7]  14.61,88.27 240 top
U$44  [VCC1]  26.04,77.15 300 top
U$45  [GND2]  27.78,73.66 300 top
U$46  [DO7]  29.84,70.33 300 top
U$47  [VCC1]  74.3,87.15 120 top
U$48  [VCC1]  86.84,85.88 120 top
U$49  [GND2]  72.55,90.65 120 top
U$50  [GND2]  85.09,89.06 120 top
U$51  [DI6]  70.33,94.46 120 top
U$52  [DO7]  83.18,92.23 120 top
U$53  [DO7]  81.44,69.22 60 top
U$54  [VCC1]  67.94,66.2 60 top
U$55  [GND2]  70.48,70.48 60 top
U$56  [GND2]  83.03,72.23 60 top
U$57  [DI6]  72.39,74.45 60 top
U$58  [VCC1]  84.77,75.09 60 top
U$59  [SDA4]  26.83,59.53 0 top
U$60  [SCL5]  30.64,59.53 0 top
U$62  [IN3]  23.65,59.37 0 top
Y1  53.24,84.62 0 top

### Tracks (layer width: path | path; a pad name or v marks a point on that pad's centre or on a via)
3.3V  (via drill 0.38)
  Top 0.178: U2.5 55.72,87.32 56.52,86.52 58.42,86.52 58.58,86.52 | U1.17 40.45,79.49 C4.1 40.41,78.83 40.32,78.74 35.08,78.74 33.84,79.98 | 33.84,79.98 33.82,80.02 | J56.P$1 33.52,79.98 33.84,79.98 | 30.86,77.72 J34.P$1 | 43.96,63.75 J73.P$1 | 43.67,60.99 J17.P$1 | 61.65,73.57 R1.2
  Top 0.203: 18.41,94.13 D31.1 23.33,94.13 24.34,95.15 C22.1 29.84,96.68 31.81,94.72 | 18.41,94.13 16.51,94.13 16.48,94.17 16.48,94.25 16.28,94.46 J44.P$1 | 18.41,94.13 18.41,84.61 17.57,83.77 D32.1 13.76,83.77 13.49,83.5 13.49,77.31 | C23.1 22.7,72.71 22.21,73.2 D33.1 18.72,73.2 v17.62,74.3 17.14,74.77 17.14,77.31 C21.1 13.49,77.31 | 13.49,77.31 13.49,76.84 12.86,76.2 J45.P$1 9.68,74.77 v9.53,74.77 | J47.P$1 71.93,88.13 72.06,88.13 72.24,87.95 76.36,87.95 76.76,88.34 | C25.1 84.61,78.42 85.72,77.31 | 86.52,79.38 86.52,80.01 86.04,80.49 84.95,80.49 D5.1 83.21,80.62 82.39,81.44 82.39,94.62 80.33,96.68 C24.1 77.37,90.96 | 86.52,79.38 86.52,78.11 85.72,77.31 | 77.37,90.96 77.37,88.96 76.76,88.34 | D2.1 77.38,90.95 77.37,90.96 | D6.1 79.08,70.01 77.37,70.01 | 77.37,70.01 C26.1 77.31,66.83 76.83,66.52 69.91,66.52 67.82,68.61 67.7,68.72 J7.P$1 | J52.P$1 87.63,79.85 87.15,79.38 86.52,79.38 | 77.37,70.01 77.37,75.41 | 77.37,75.41 77.37,76.26 77.79,76.68 77.79,87.31 76.76,88.34 | 77.37,75.41 77.33,75.45 | J57.P$1 87.15,75.88 85.72,77.31 | J62.P$1 72.07,54.77 | 72.07,54.77 74.3,54.77 | 74.3,54.77 J60.P$1 | D1.A 72.07,54.77 | 74.3,54.77 J64.P$1 v74.3,63.5 | 49.85,15.72 J68.P$1 | 52.23,15.72 49.85,15.72 | 52.23,15.72 53.02,15.72 J66.P$1 | 49.85,15.72 D3.A | J70.P$1 52.39,15.88 52.23,15.72 | U4.P$6 29.37,53.67 | 29.37,53.67 26.67,53.67 | 26.67,53.67 U4.P$5 25.07,53.67 23.81,54.93 J1.P$1 v21.27,55.56 | C16.1 26.83,50.8 26.67,50.96 26.67,53.67 | U4.P$10 29.63,55.67 29.37,55.4 29.37,53.67 | U5.5 42.23,34.61 41.7,35.14 R9.2 40.8,36.04 40.64,36.2 40.64,38.89 41.59,39.85 | U6.5 49.59,34.51 50.06,34.98 | 50.06,34.98 51.28,34.98
  Top 0.203: 51.28,34.98 C9.1 54.19,34.98 55.25,36.04 IC1.1 57.79,36.04 58.21,36.46 C18.2 | R2.2 51.59,37.31 51.28,36.99 51.28,34.98 | C8.1 45.66,87 | J30.P$1 42.86,41.12 41.59,39.85 | 50.06,34.98 50.01,35.04 50.01,38.1 48.9,39.21 42.23,39.21 41.59,39.85 | R10.2 55.29,54.29 54.64,53.64 49.06,53.64 48.72,53.98 48.72,55.81 | 48.72,55.81 U7.8 | 48.72,55.81 U7.8 48.25,56.27 47.92,56.27 R29.2 46.99,57.47 J17.P$1 43.66,63.02 43.96,63.75 | 43.67,60.99 v40.63,57.95 40.48,57.8 J28.P$1 | 49.85,69.73 R8.2 48.85,69.69 R6.2 44.61,69.69 43.97,69.06 J73.P$1 | 49.85,69.73 50.55,69.73 C1.1 57.79,69.64 | 49.85,69.73 49.85,72.39 49.69,72.55 49.69,74.38 U1.36 49.58,79.44 49.53,79.49 | 58.42,86.52 63.18,86.52 64.86,84.84 v64.86,78.58 64.86,74.87 63.64,73.64 R1.2 57.79,69.85 57.79,69.64 | J76.P$1 59.27,69.64 57.79,69.64 | U1.44 49.53,79.49 | U1.17 v45.09,79.49 49.53,79.49 | J70.P$1 52.07,21.91 | J57.P$1 88.42,74.93 | L1.1 45.66,87 | 45.66,87 v44.45,87 | v90.09,74.59 87.88,75.88 J57.P$1 | J70.P$1 v52.23,24.29 | J56.P$1 32.23,79.06 31.75,78.74 31.43,78.58 30.86,77.72
  Route15 0.203: 40.49,45.4 J28.P$1 40.48,45.39 40.41,45.32 40.41,44.94 40.48,44.87 40.48,44.45 40.96,43.97 42.39,43.97 43.02,43.34 43.02,43.02 42.96,42.96 42.96,42.57 43.18,42.36 J30.P$1 | J7.P$1 66.72,69.7 65.98,69.7 65.52,70.17 65.09,70.17
  Bottom 0.178: JP5.1 60.67,78.58 64.61,78.58
  Bottom 0.203: v17.62,74.3 18.1,73.82 20.48,76.2 J34.P$1 | J47.P$1 71.91,88.11 | 64.61,78.58 v64.86,78.58 | J30.P$1 43.02,41.28 43.02,43.34 42.39,43.97 40.96,43.97 40.48,44.45 J28.P$1
  pour Route15: 13.02,104.77 86.84,104.77 99.85,82.23 50.01,0 0,82.23
!RESET
  Top 0.178: 56.62,75.41 56.58,75.37 | 56.58,75.37 S1.4 55.88,77.02 JP5.10 55.37,77.49 U1.40 | 56.58,75.37 S1.3 61.54,75.37 R1.1
A3  (via drill 0.38)
  Top 0.178: J10.P$1 35.66,87.05 39.85,82.87
  Top 0.203: IC1.3 54.77,33.5 v54.61,33.34 | 39.85,82.87 42.7,82.87 43.82,81.76 45.4,81.76 45.58,81.94 U1.9
  Route2 0.203: v89.22,83.98 85.64,80.4 65.18,80.4 61.59,83.98 45.24,83.98 42.17,87.05 J10.P$1
  Bottom 0.203: v54.61,33.34 54.61,39.05 | 54.61,39.05 J37.P$1 | 54.61,39.05 69.69,39.05 74.93,44.29 74.93,48.26 82.87,56.2 82.87,59.69 88.74,65.56 88.74,72.23 96.2,79.69 96.2,83.5 94.46,85.25 90.33,85.25 89.22,84.14 v89.22,83.98
AUD
  Top 0.203: R3.1 C17.2 40.96,31.06 40.96,29.53 41.59,28.89 42.23,28.89 | U5.1 42.23,28.89 | 42.23,28.89 42.23,27.94 43.02,27.15 R13.1
D2  (via drill 0.38)
  Top 0.178: U1.23 40.28,76.49 39.48,75.69 39.46,75.71 v39.46,75.76
  Top 0.203: D2.4 72.72,90.95 69.21,94.46 J53.P$1
  Bottom 0.178: v39.46,75.76 39.46,75.63 | 55.35,70.25 56.5,69.1 56.5,69.07 56.67,68.9 J14.P$1
  Bottom 0.203: v39.46,75.76 45.36,75.76 46.51,74.61 51.59,74.61 54.45,71.76 54.45,71.16 55.35,70.25 | J14.P$1 56.67,63.98 56.99,63.66 60.33,63.66 61.28,63.98 61.75,64.93 62.39,66.04 64.29,69.85 67.79,76.04 68.26,76.68 68.9,77.15 69.69,77.15 J42.P$1 72.71,77.31 74.93,79.85 76.99,81.92 76.99,83.98 73.66,87.31 73.66,93.19 72.39,94.46 68.43,94.46 68.25,94.63 J53.P$1
D3
  Top 0.178: U1.14 36.8,80.99 33.79,84 33.79,84.13 33.62,84.3 J23.P$1
  Top 0.203: U4.P$4 25.36,54.17 25.08,54.45 25.08,60.8 J22.P$1
  Route2 0.203: J22.P$1 24.92,77.15 23.49,78.58 23.49,82.89 25.73,85.12 25.74,85.11 28.14,85.11 28.16,85.09 28.87,85.09 28.95,85.11 29.01,85.08 29.18,85.08 29.33,84.93 32.23,84.93 J23.P$1 33.31,84.3
D5  (via drill 0.38)
  Top 0.178: U1.24 41.38,75.99 39.37,73.98 39.37,72.23 38.58,71.44 J3.P$1
  Top 0.203: R29.1 46.94,55.46 46.94,53.67 | U7.5 51.64,55.79 51.64,54.95 52.1,54.49 v52.75,54.49 53.51,54.49 53.82,54.8 C13.1 | C12.A 46.94,53.67 | 46.94,53.67 47.95,53.67 49.16,52.45 50.95,52.45 v50.96,52.46
  Route2 0.203: J24.P$1 53.18,44.45 52.71,43.97 26.19,43.97 24.45,47.15 15.88,62.55 14.13,62.71 v14.29,62.71
  Route15 0.203: v14.29,62.71 16.83,63.5 24.29,63.5 24.92,63.82 24.92,77.15 23.18,78.9 23.02,83.19 25.56,85.09 25.72,85.25 28.42,85.14 28.43,85.13 28.49,85.13 28.54,85.11 28.63,85.13 29.69,85.09 29.69,84.61 28.89,82.87 30.32,78.9 35.24,70.64 36.04,70.17 J3.P$1
  Bottom 0.203: J24.P$1 53.18,52.4 | 53.18,52.4 53.18,54.19 52.88,54.49 v52.75,54.49 | v50.96,52.46 53.12,52.46 53.18,52.4
D6  (via drill 0.38)
  Top 0.178: 34.37,71.19 J26.P$1 29.3,69.69 28.28,70.71 28.28,73.44 26.7,75.02 26.7,78.37 23.63,81.44 23.63,86.98 25.4,88.75
  Top 0.203: D31.4 24.44,94.13 24.13,93.82 24.13,90.01 25.4,88.75 26.04,88.11 J32.P$1 | U1.29 46.04,74.45 46.04,73.18 44.61,71.76 41.43,71.76 41.27,71.91 v41.12,71.91 | J18.P$1 35.73,72.94 34.9,72.36 34.37,71.19
  Bottom 0.203: v41.12,71.91 38.58,74.45 37.15,74.45 37.14,74.44 | 37.14,74.44 37.14,74.31 | J18.P$1 37.14,74.44
D7  (via drill 0.38)
  Top 0.203: U7.2 49.68,58.57 50.32,59.21 54.77,59.21 55.25,58.74 55.25,58.22 55.29,58.17 R10.1 55.89,57.33 56.47,56.76 56.47,47.3 56.36,47.19 J40.P$1 56.36,44.13 55.88,43.82 28.73,43.82 23.65,46.83 16.19,60.64 v17.14,62.55 | J5.P$1 40.96,68.58 41.43,69.06 42.67,69.06 46.58,72.97 U1.30
  Bottom 0.203: v17.14,62.55 17.14,63.34 17.67,63.34 17.72,63.37 17.83,63.34 38.26,63.34 38.89,63.98 38.89,64.61 37.94,65.56 37.94,67.47 J5.P$1
D8  (via drill 0.38)
  Top 0.203: IC1.4 56.1,32.07 v51.12,32.07 | U1.11 44.58,84.17 38.26,90.49 38.26,91.84 38.57,92.37 38.44,92.37 J8.P$1
  Bottom 0.203: J35.P$1 51.12,40.8 51.12,38.89 | 51.12,38.89 v51.12,32.07 | J8.P$1 36.24,93.79 36.2,93.82 36.2,94.99 36.24,94.99 | 51.12,38.89 34.45,38.89 33.5,37.94 32.23,37.31 32.07,37.15 30.64,37.15 28.57,40.48 4.45,81.76 13.34,98.9 14.92,100.49 38.26,100.49 38.73,100.01 36.24,94.99 | 36.24,94.98 36.24,94.99
D9  (via drill 0.38)
  Top 0.203: U1.12 44.08,83.71 37.94,89.85 37.16,89.85 36.98,89.67 36.8,89.85 J9.P$1 | J36.P$1 59.05,40.48 63.98,40.48 65.88,38.58 65.88,37.62 63.02,34.77 IC1.7 60.17,34.77 60.01,34.61 v59.85,34.61
  Route15 0.203: v59.85,34.61 62.71,34.61 63.98,33.34 66.04,33.34 70.48,37.78 70.48,41.28 79.53,50.32 79.53,55.56 86.68,62.71 86.68,67.63 94.3,75.25 94.3,84.77 93.66,85.25 92,85.25 91.98,85.22 91.92,85.22 91.88,85.2 91.77,85.22 90.87,85.22 90.82,85.2 90.72,85.22 90.61,85.22 90.58,85.25 90.33,85.25 90.33,83.66 89.38,82.71 87.95,82.71 85.62,80.38 65.35,80.38 61.91,83.82 v41.91,83.82
  Bottom 0.203: v41.91,83.82 41.91,85.88 37.94,89.85 37.16,89.85 36.98,89.67 36.85,89.67 J9.P$1
DO
  Top 0.203: D33.2 16.81,70 J41.P$1
  Bottom 0.203: J54.P$1 16.19,84.21 16.19,70.09 16.5,69.55 16.37,69.55 J41.P$1
DOUT  (via drill 0.38)
  Top 0.203: J48.P$1 83.5,93.98 v83.5,86.36 | v78.58,75.09 78.58,73.71 79,73.29 | 79,73.29 D6.2 | J50.P$1 83.66,69.69 80.06,73.29 79,73.29
  Bottom 0.203: v83.5,86.36 78.58,81.44 v78.58,75.09
GND  (via drill 0.38)
  Top 0.152: U4.P$8 31.71,54.67 33.02,55.98 J20.P$1
  Top 0.178: J33.P$1 32.41,74.47 J6.P$1 | 47.21,61.18 J19.P$1
  Top 0.203: J19.P$1 46.83,63.18 arc-28 46.99,63.82 arc49 J11.P$1 | v48.91,73.19 48.9,73.18 48.9,73.52 49.08,73.71 U1.35 | J63.P$1 69.69,63.66 | J61.P$1 64.29,56.67 | J59.P$1 79.85,56.83 | 87.88,71.29 85.74,72.71 J58.P$1 | J65.P$1 47.15,24.29 | J20.P$1 34.61,56.67 35.4,56.04 | J55.P$1 67.61,74.28
  Bottom 0.203: J65.P$1 46.99,21.75 | J29.P$1 43.66,44.45 44.45,43.66 46.36,43.66 46.99,43.02 J31.P$1 | v48.91,73.19 48.92,73.18
  other vias: 75.88,77.15 73.5,84.77 76.52,86.68 89.38,81.28 49.69,22.38 47.62,18.1 51.44,12.86 47.94,12.86 70.17,52.23 73.82,51.75 23.02,59.37 25.72,52.7 30.16,50.64 34.77,59.21 36.83,51.28 43.18,54.45 58.42,55.72 62.87,50.01 51.28,83.03 58.42,84.93 40.01,85.25 36.99,83.82 58.42,87.95 35.56,80.49 36.99,76.36 46.51,80.96 47.62,81.12 48.9,92.55 51.12,73.18 44.45,77.63 46.2,76.83 35.56,49.05 37.47,53.66 62.71,53.82 63.98,47.31 42.23,50.8 38.89,40.8 36.35,36.67 52.86,40.16 65.09,41.43 52.71,29.37 51.91,58.42 81.76,56.04 85.09,64.13 93.19,78.42 51.59,48.1 28.57,42.54 18.1,61.12 10.64,68.42 15.88,89.38 20.95,87.47 28.42,93.5 11.91,82.87 29.21,67.15 20.8,66.67 40.48,95.09 63.5,84.61 53.82,75.72 57.63,68.42 46.2,68.1 19.21,96.36
  pour Top: 13.02,104.77 86.84,104.77 99.85,82.23 50.01,0 0,82.23
  pour Bottom: 0.16,82.23 13.02,104.77 86.68,104.77 86.84,104.77 99.85,82.23 50.01,0
  pour Route2: 13.02,104.77 86.84,104.77 99.85,82.23 50.01,0 0,82.07 0,82.23
ID  (via drill 0.38)
  Top 0.178: R5.2 60.38,80.8 v62.07,80.8
  Top 0.203: U3.1 47.64,89.84 47.47,90.01 47.47,90.81 | 47.47,90.81 47.47,94.93 47.62,95.09 48.42,95.09 | 48.42,95.09 49.21,95.09 49.5,94.81 JP3.ID1 | U3.2 47.48,90.79 47.47,90.81 | R4.1 56.36,97.31 55.88,97.79 v55.25,97.79 48.58,97.79 48.42,97.63 48.42,95.09
  Bottom 0.178: v62.07,80.8 62.07,88.42 57.63,92.87 57.63,97 56.83,97.79 v55.25,97.79 54.93,97.79
N$1
  Top 0.406: JP3.VBUS1 51.45,92.22 51.75,91.92 F1.1
N$2
  Top 0.178: U1.1 49.58,82.18 49.85,81.92 53.18,81.92 54.16,82.89 C5.2 54.16,84.28 Y1.P$2
N$3
  Top 0.203: U6.1 47.19,33.53 48.26,34.61 C19.1
N$4
  Top 0.178: U1.2 49.08,84.32 49.38,84.62 Y1.P$1 52,85.71 C6.1
N$5
  Top 0.203: U7.3 U7.4
N$6
  Top 0.203: C17.1 41.33,32.39 43.97,32.39 44.13,32.54 44.13,32.55 U5.4 44.29,33.69 44.29,34.61 44.93,35.24 46.3,35.24 R12.1 46.36,34.13 45.94,33.71 R13.2
N$7  (via drill 0.38)
  Top 0.178: F1.2 51.75,87.63 52.07,87.31 54.13,87.31 54.29,87.47 v54.29,87.63
  Top 0.203: Q2.3 43.02,96.04 v43.66,96.68
  Bottom 0.178: 52.71,87.63 v54.29,87.63
  Bottom 0.203: v43.66,96.68 43.66,94.77 48.08,90.35 48.29,90.35 51,87.63 52.71,87.63
N$8
  Bottom 0.203: J74.P$1 59.53,57.63 J21.P$1
N$9
  Top 0.203: Q2.1 43.97,91.79 44.02,91.74 | 44.02,91.74 R7.1 | U3.4 44.02,91.74
N$10
  Top 0.203: R12.2 C19.2
N$11  (via drill 0.38)
  Top 0.203: R11.2 43.4,36.99 | R9.1 43.4,36.99 | 43.4,36.99 v44.61,36.99 | v44.77,29.37 44.45,29.37 44.13,29.69 U5.3 | C20.1 40.32,35.3 40.32,34.61 v40.48,34.61
  Bottom 0.203: v44.61,36.99 44.77,36.83 44.77,34.45 | 44.77,34.45 v44.77,29.37 | v40.48,34.61 40.64,34.45 44.77,34.45
N$12
  Top 0.203: R15.2 71.23,56.95 D1.C
N$13  (via drill 0.38)
  Top 0.203: U4.P$1 25.72,56.31 25.72,56.52 v25.88,56.67 | v30.8,52.39 C15.1
  Bottom 0.203: v25.88,56.67 27.15,55.4 27.15,52.55 27.3,52.39 v30.8,52.39
N$14
  Top 0.203: D31.2 22.25,90.93 22.54,90.65 22.54,84.3 22.02,83.77 D32.4 20.53,83.66
N$15
  Top 0.203: R17.2 49.04,18.18 D3.C
N$16
  Top 0.203: D32.2 17.7,80.57 19.68,78.58 24.76,78.58 26.04,77.31 26.04,76.68 26.07,76.64 D33.4
N$17
  Top 0.203: IC1.5 61.86,31.38 61.12,30.64 61.12,29.21 60.48,28.58 55.88,28.58 54.29,26.99 C14.2
N$18  (via drill 0.38)
  Top 0.203: R3.2 38.73,34.29 38.42,34.61 v38.1,34.61 | v49.69,26.83 51.22,26.83 C14.1
  Bottom 0.203: v38.1,34.61 45.88,26.83 v49.69,26.83
N$19
  Top 0.203: IC1.6 60.17,33.5 59.91,33.24 C10.1
N$20
  Top 0.203: IC1.8 61.86,37.15 62.36,37.65 C11.1 | C11.1 | R2.1 55.25,37.31 56.99,39.05 62.07,39.05 62.39,38.74 C11.1
N$21
  Top 0.178: 64.13,87.31 64.2,87.31 64.23,87.28 64.23,87.25 64.13,87.15 61.12,87.15
  Top 0.203: J71.P$1 64.13,87.31 63.82,87.31 | S2.3 60.99,89.41 60.17,88.58 60.17,87.47 60.48,87.15 61.12,87.15
N$22
  Top 0.203: D5.4 81.09,80.62 81.44,80.96 81.44,93.5 80.79,94.15 D2.2
N$23  (via drill 0.38)
  Top 0.203: D6.4 74.11,70.17 v75.88,70.17 | v86.68,84.77 86.68,84.14 86.36,83.82 D5.2
  Bottom 0.203: v75.88,70.17 77.47,70.17 81.91,74.61 81.91,80.01 v86.68,84.77
N$24
  Top 0.203: U4.P$9 31.68,55.17 31.91,55.4 31.91,55.88 29.96,57.83 JP2.1
N$25  (via drill 0.38)
  Top 0.203: U4.P$7 32.1,54.17 v32.23,54.29
  Bottom 0.203: JP2.2 26.99,58.9 27.15,59.06 31.75,59.06 31.91,58.9 31.91,58.1 31.75,57.94 31.75,56.52 32.23,56.04 v32.23,54.29
SCL  (via drill 0.38)
  Top 0.178: J15.P$1 53.34,60.96 53.69,61.31
  Top 0.203: U4.P$2 27.39,55.17 v27.94,55.72 | v31.11,58.26 31.11,59.69 J4.P$1 | U7.7 49.68,54.45 49.69,54.44 | 49.69,54.44 | 49.69,54.44 v49.67,54.42 | U1.32 47.62,74.45 47.62,73.18 v48.02,72.79 48.9,71.91 R8.1 | 53.34,61.6 arc-50 53.34,60.96 | J15.P$1 53.13,60.85 53.13,62.88 53.5,64.35 53.5,64.45 | 53.5,64.45 53.5,64.61 | J38.P$1 53.5,64.45
  Route15 0.203: J4.P$1 32.39,63.34 32.47,63.43 52.79,63.43 53.34,63.5 53.54,64.17 J38.P$1
  Bottom 0.203: v27.94,55.72 28.57,56.36 30.64,56.36 31.11,56.83 v31.11,58.26 | J15.P$1 52.85,60.47 52.85,57.6 v49.67,54.42 50.01,54.08 J13.P$1 | J4.P$1 32.39,62.11 | v48.02,72.79 48.02,71.75 J38.P$1
SDA  (via drill 0.38)
  Top 0.178: 50.49,61.29 50.09,60.88 J16.P$1
  Top 0.203: U4.P$3 28.63,54.67 28.89,54.93 28.89,56.2 28.26,56.83 28.26,60.64 J2.P$1 | U7.1 48.71,59.18 49.76,60.23 49.76,60.56 J16.P$1 | U1.31 47.08,72.3 47.18,72.2 R6.1 46.15,71.39 v46.04,71.28 | 50.09,60.88 arc-51 50.16,63.02 arc55 50.16,63.18 50.16,63.95 50.19,63.97 50.19,64.57 J12.P$1
  Route2 0.203: J2.P$1 28.57,63.34 28.68,63.44 49,63.44 49.7,63.43 50.16,63.82 50.16,66.04 J12.P$1
  Bottom 0.203: J39.P$1 46.83,57.63 J16.P$1 | J12.P$1 50.32,66.99 v46.04,71.28
SWCLK
  Top 0.178: U1.45 53.8,79.99 56.99,83.19 62.55,83.19 62.87,82.87 62.87,77.47 61.91,76.52 59.53,76.52 59.2,76.85 JP5.4
SWDIO  (via drill 0.38)
  Top 0.178: U1.46 53.34,80.49 56.67,83.82 62.55,83.82 63.66,82.71 v63.66,77.47
  Bottom 0.178: JP5.2 60.52,77.47 v63.66,77.47
USB_D+  (via drill 0.38)
  Top 0.203: JP3.D+1 50.15,92.53 49.69,92.08 49.69,87.47 v49.53,87.31 | U1.34 48.58,75.41 48.9,75.72 48.9,77.79 v48.58,78.11
  Bottom 0.203: v49.53,87.31 49.53,78.9 48.58,77.95 v48.58,78.11
USB_D-  (via drill 0.38)
  Top 0.203: JP3.D-1 50.8,92.39 50.32,91.92 v50.32,86.36 | v48.1,76.2 48.1,74.51 U1.33
  Bottom 0.203: v50.32,86.36 50.32,78.58 48.1,76.36 v48.1,76.2
USB_HOST_EN
  Top 0.178: U1.41 53.86,77.99 54.62,78.75 54.62,79.1 56.17,80.65 R5.1
VDDANA
  Top 0.178: U1.6 47.08,83.91 47.36,84.19 C3.1
  Top 0.203: L1.2 48.1,86.36 48.26,86.2 48.26,85.25 48.1,85.09 C3.1
VDDCORE
  Top 0.178: U1.43 53.75,78.99 56.83,82.07 C2.1
VIN  (via drill 0.38)
  Top 0.178: S2.2 57.31,92.01
  Top 0.203: U3.5 45.66,89.98 R7.2 v42.55,89.98 42.42,89.98 42.07,90.33 Q2.2 | U2.3 53.82,91.12 53.98,90.96 55.56,90.96 55.72,91.12 55.72,91.13 U2.1 55.72,92.71 55.88,92.87 56.52,92.87 | C7.1 57.31,92.01 57.31,92.71 57.15,92.87 56.52,92.87 | R4.2 56.52,94.77 v56.52,93.35 56.52,92.87
  Bottom 0.178: v42.55,89.98 48.13,89.98 51.59,86.52 55.56,86.52 56.52,87.47 v56.52,93.35 56.52,93.66

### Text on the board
tPlace: + | + | + | - | - | - | - | - | + | + | +

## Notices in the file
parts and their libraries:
SparkFun-Aesthetics: Licensing: Creative Commons ShareAlike 4.0 International - https://creativecommons.org/licenses/by-sa/4.0
